FUNCTION "Gest Automatico" : VOID
TITLE =GESTIONE AUTOMATICO
AUTHOR : MassimoZ
VERSION : 0.1

BEGIN
NETWORK
TITLE ======== Automatico Barra 1 =======

NETWORK
TITLE =Aux Emergenze Macchine Barra 1 Intervenuta
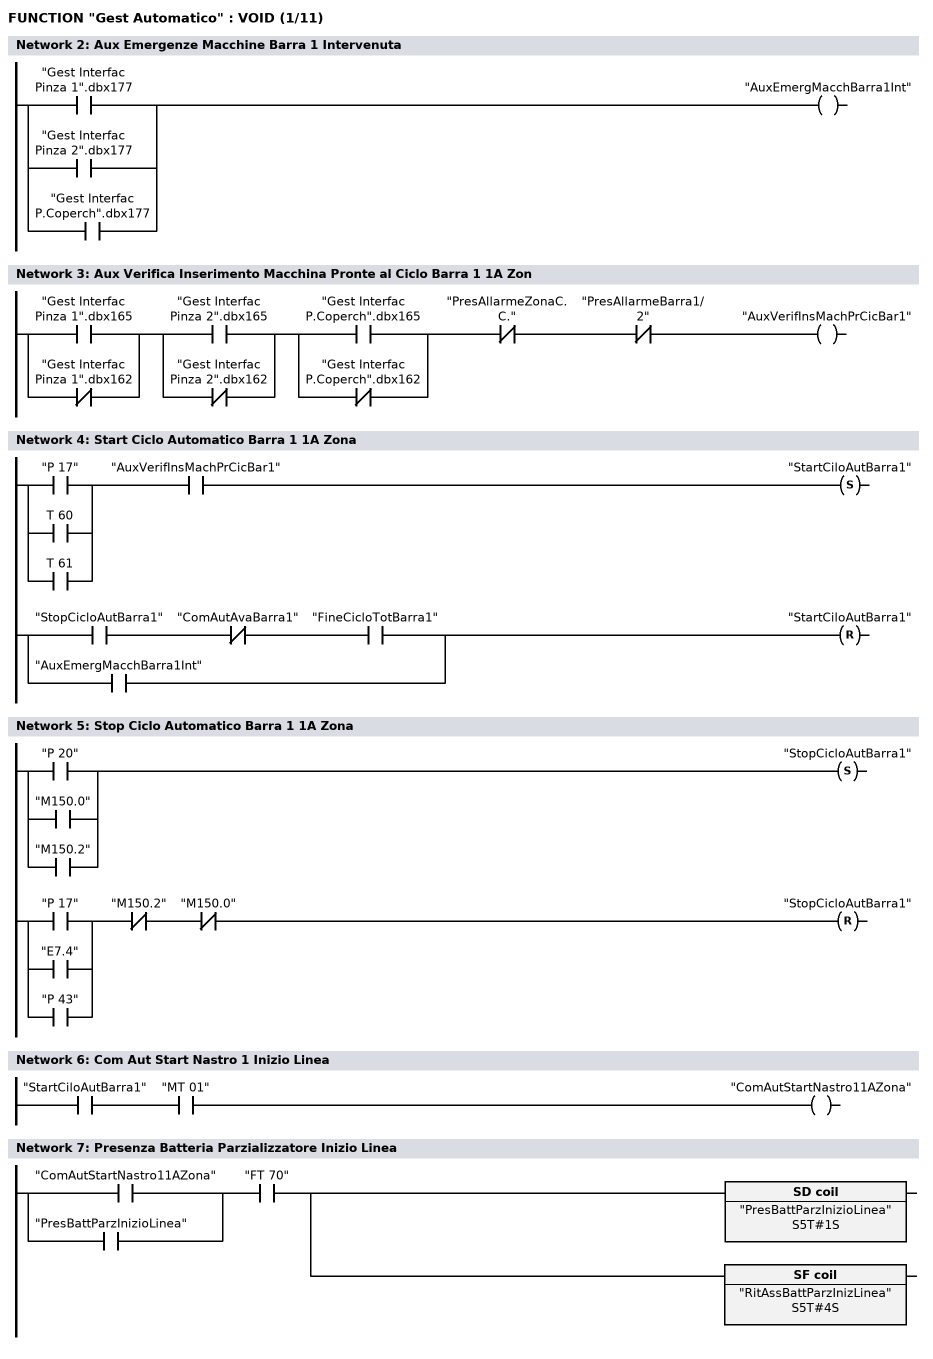
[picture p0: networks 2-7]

      O     "Gest Interfac Pinza 1".dbx177;
      O     "Gest Interfac Pinza 2".dbx177;
      O     "Gest Interfac P.Coperch".dbx177;
      =     "AuxEmergMacchBarra1Int";
NETWORK
TITLE =Aux Verifica Inserimento Macchina Pronte al Ciclo Barra 1 1A Zon

      U(    ;
      O     "Gest Interfac Pinza 1".dbx165;
      ON    "Gest Interfac Pinza 1".dbx162;
      )     ;
      U(    ;
      O     "Gest Interfac Pinza 2".dbx165;
      ON    "Gest Interfac Pinza 2".dbx162;
      )     ;
      U(    ;
      O     "Gest Interfac P.Coperch".dbx165;
      ON    "Gest Interfac P.Coperch".dbx162;
      )     ;
      UN    "PresAllarmeZonaC.C.";
      UN    "PresAllarmeBarra1/2";
      =     "AuxVerifInsMachPrCicBar1";
NETWORK
TITLE =Start Ciclo Automatico Barra 1 1A Zona

      U(    ;
      O     "P 17";
      O     T     60;
      O     T     61;
      )     ;
      U     "AuxVerifInsMachPrCicBar1";
      S     "StartCiloAutBarra1";
      U(    ;
      U     "StopCicloAutBarra1";
      UN    "ComAutAvaBarra1";
      U     "FineCicloTotBarra1";
      O     "AuxEmergMacchBarra1Int";
      )     ;
      R     "StartCiloAutBarra1";
      NOP   0;
NETWORK
TITLE =Stop Ciclo Automatico Barra 1 1A Zona

      U(    ;
      O     "P 20";
      O     "M150.0";
      O     "M150.2";
      )     ;
      S     "StopCicloAutBarra1";
      U(    ;
      O     "P 17";
      O     "E7.4";
      O     "P 43";
      )     ;
      UN    "M150.2";
      UN    "M150.0";
      R     "StopCicloAutBarra1";
      NOP   0;
NETWORK
TITLE =Com Aut Start Nastro 1 Inizio Linea

      U     "StartCiloAutBarra1";
      U     "MT 01";
      =     "ComAutStartNastro11AZona";
NETWORK
TITLE =Presenza Batteria Parzializzatore Inizio Linea

      U(    ;
      O     "ComAutStartNastro11AZona";
      O     "PresBattParzInizioLinea";
      )     ;
      U     "FT 70";
      L     S5T#1S;
      SE    "PresBattParzInizioLinea";
      L     S5T#4S;
      SA    "RitAssBattParzInizLinea";
NETWORK
TITLE =Verifica Mancanza Batteria su Parzializzatore Inizio Linea
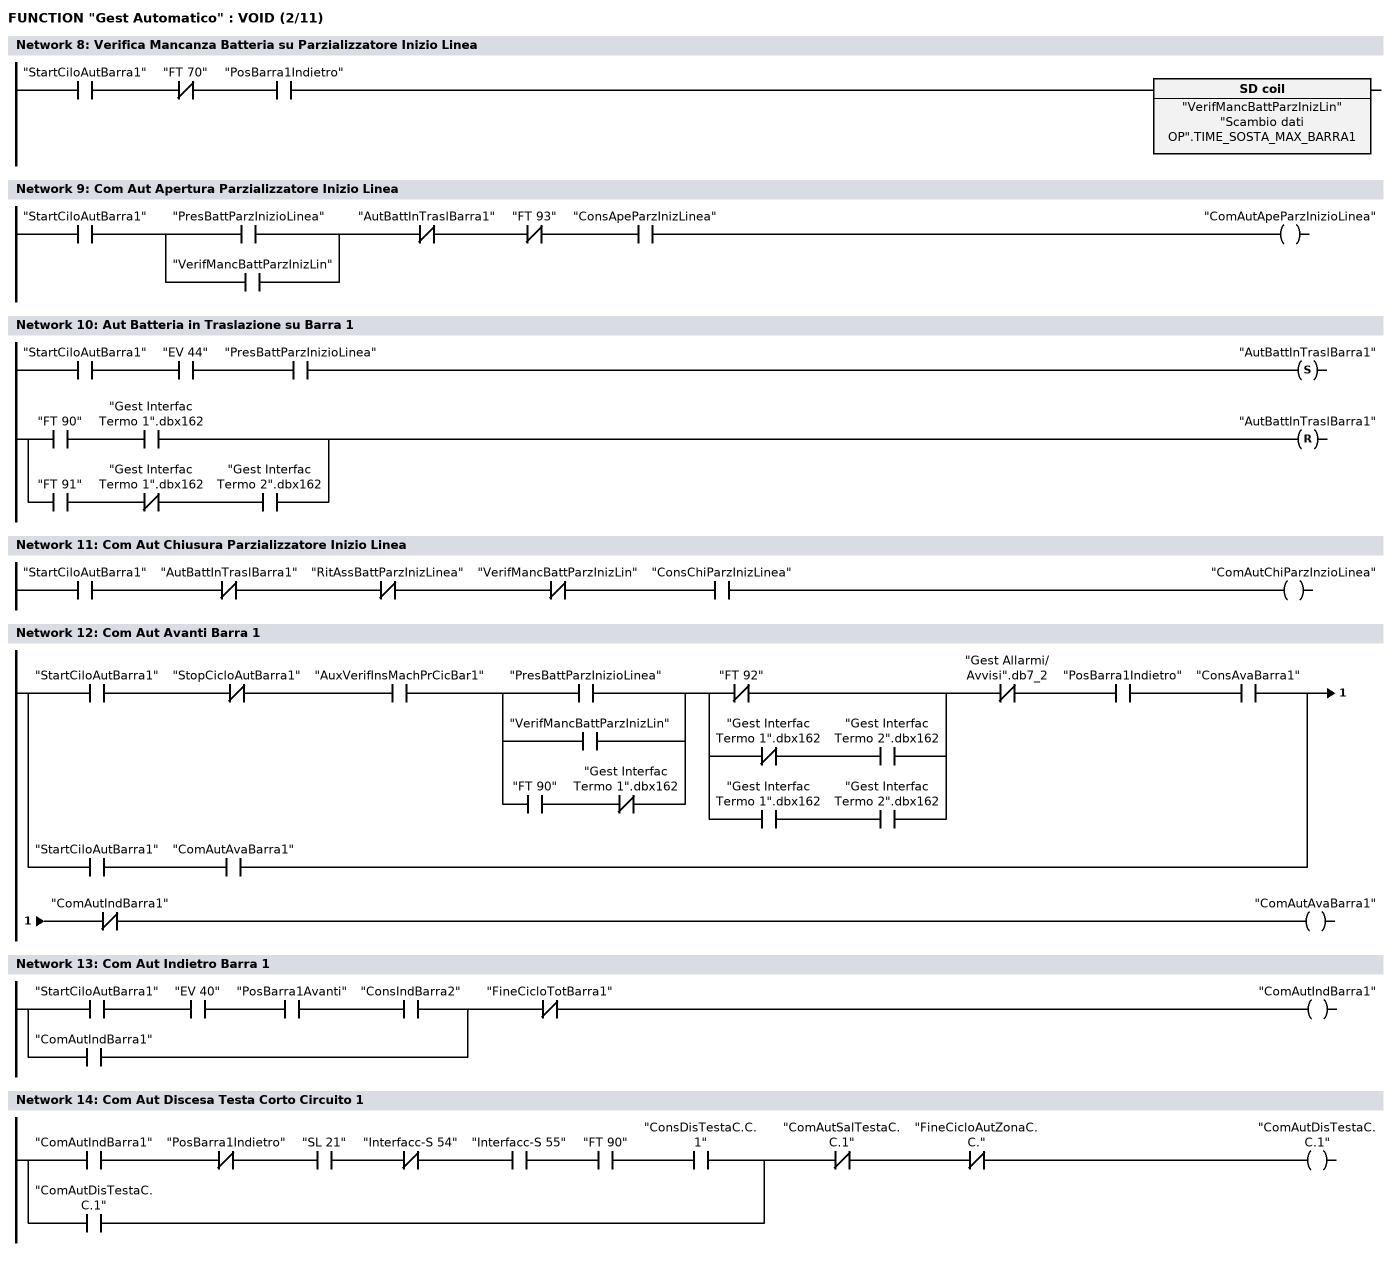
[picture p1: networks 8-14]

      U     "StartCiloAutBarra1";
      UN    "FT 70";
      U     "PosBarra1Indietro";
      L     "Scambio dati OP".TIME_SOSTA_MAX_BARRA1;
      SE    "VerifMancBattParzInizLin";
NETWORK
TITLE =Com Aut Apertura Parzializzatore Inizio Linea

      U     "StartCiloAutBarra1";
      U(    ;
      O     "PresBattParzInizioLinea";
      O     "VerifMancBattParzInizLin";
      )     ;
      UN    "AutBattInTraslBarra1";
      UN    "FT 93";
      U     "ConsApeParzInizLinea";
      =     "ComAutApeParzInizioLinea";
NETWORK
TITLE =Aut Batteria in Traslazione su Barra 1

      U     "StartCiloAutBarra1";
      U     "EV 44";
      U     "PresBattParzInizioLinea";
      S     "AutBattInTraslBarra1";
      U(    ;
      U     "FT 90";
      U     "Gest Interfac Termo 1".dbx162;
      O     ;
      U     "FT 91";
      UN    "Gest Interfac Termo 1".dbx162;
      U     "Gest Interfac Termo 2".dbx162;
      )     ;
      R     "AutBattInTraslBarra1";
      NOP   0;
NETWORK
TITLE =Com Aut Chiusura Parzializzatore Inizio Linea

      U     "StartCiloAutBarra1";
      UN    "AutBattInTraslBarra1";
      UN    "RitAssBattParzInizLinea";
      UN    "VerifMancBattParzInizLin";
      U     "ConsChiParzInizLinea";
      =     "ComAutChiParzInzioLinea";
NETWORK
TITLE =Com Aut Avanti Barra 1

      U(    ;
      U     "StartCiloAutBarra1";
      UN    "StopCicloAutBarra1";
      U     "AuxVerifInsMachPrCicBar1";
      U(    ;
      O     "PresBattParzInizioLinea";
      O     "VerifMancBattParzInizLin";
      O     ;
      U     "FT 90";
      UN    "Gest Interfac Termo 1".dbx162;
      )     ;
      U(    ;
      ON    "FT 92";
      O     ;
      UN    "Gest Interfac Termo 1".dbx162;
      U     "Gest Interfac Termo 2".dbx162;
      O     ;
      U     "Gest Interfac Termo 1".dbx162;
      U     "Gest Interfac Termo 2".dbx162;
      )     ;
      UN    "Gest Allarmi/Avvisi".db7_2;
      U     "PosBarra1Indietro";
      U     "ConsAvaBarra1";
      O     ;
      U     "StartCiloAutBarra1";
      U     "ComAutAvaBarra1";
      )     ;
      UN    "ComAutIndBarra1";
      =     "ComAutAvaBarra1";
NETWORK
TITLE =Com Aut Indietro Barra 1

      U(    ;
      U     "StartCiloAutBarra1";
      U     "EV 40";
      U     "PosBarra1Avanti";
      U     "ConsIndBarra2";
      O     "ComAutIndBarra1";
      )     ;
      UN    "FineCicloTotBarra1";
      =     "ComAutIndBarra1";
NETWORK
TITLE =Com Aut Discesa Testa Corto Circuito 1

      U(    ;
      U     "ComAutIndBarra1";
      UN    "PosBarra1Indietro";
      U     "SL 21";
      UN    "Interfacc-S 54";
      U     "Interfacc-S 55";
      U     "FT 90";
      U     "ConsDisTestaC.C.1";
      O     "ComAutDisTestaC.C.1";
      )     ;
      UN    "ComAutSalTestaC.C.1";
      UN    "FineCicloAutZonaC.C.";
      =     "ComAutDisTestaC.C.1";
NETWORK
TITLE =Com Aut Start Corto Circuito 1
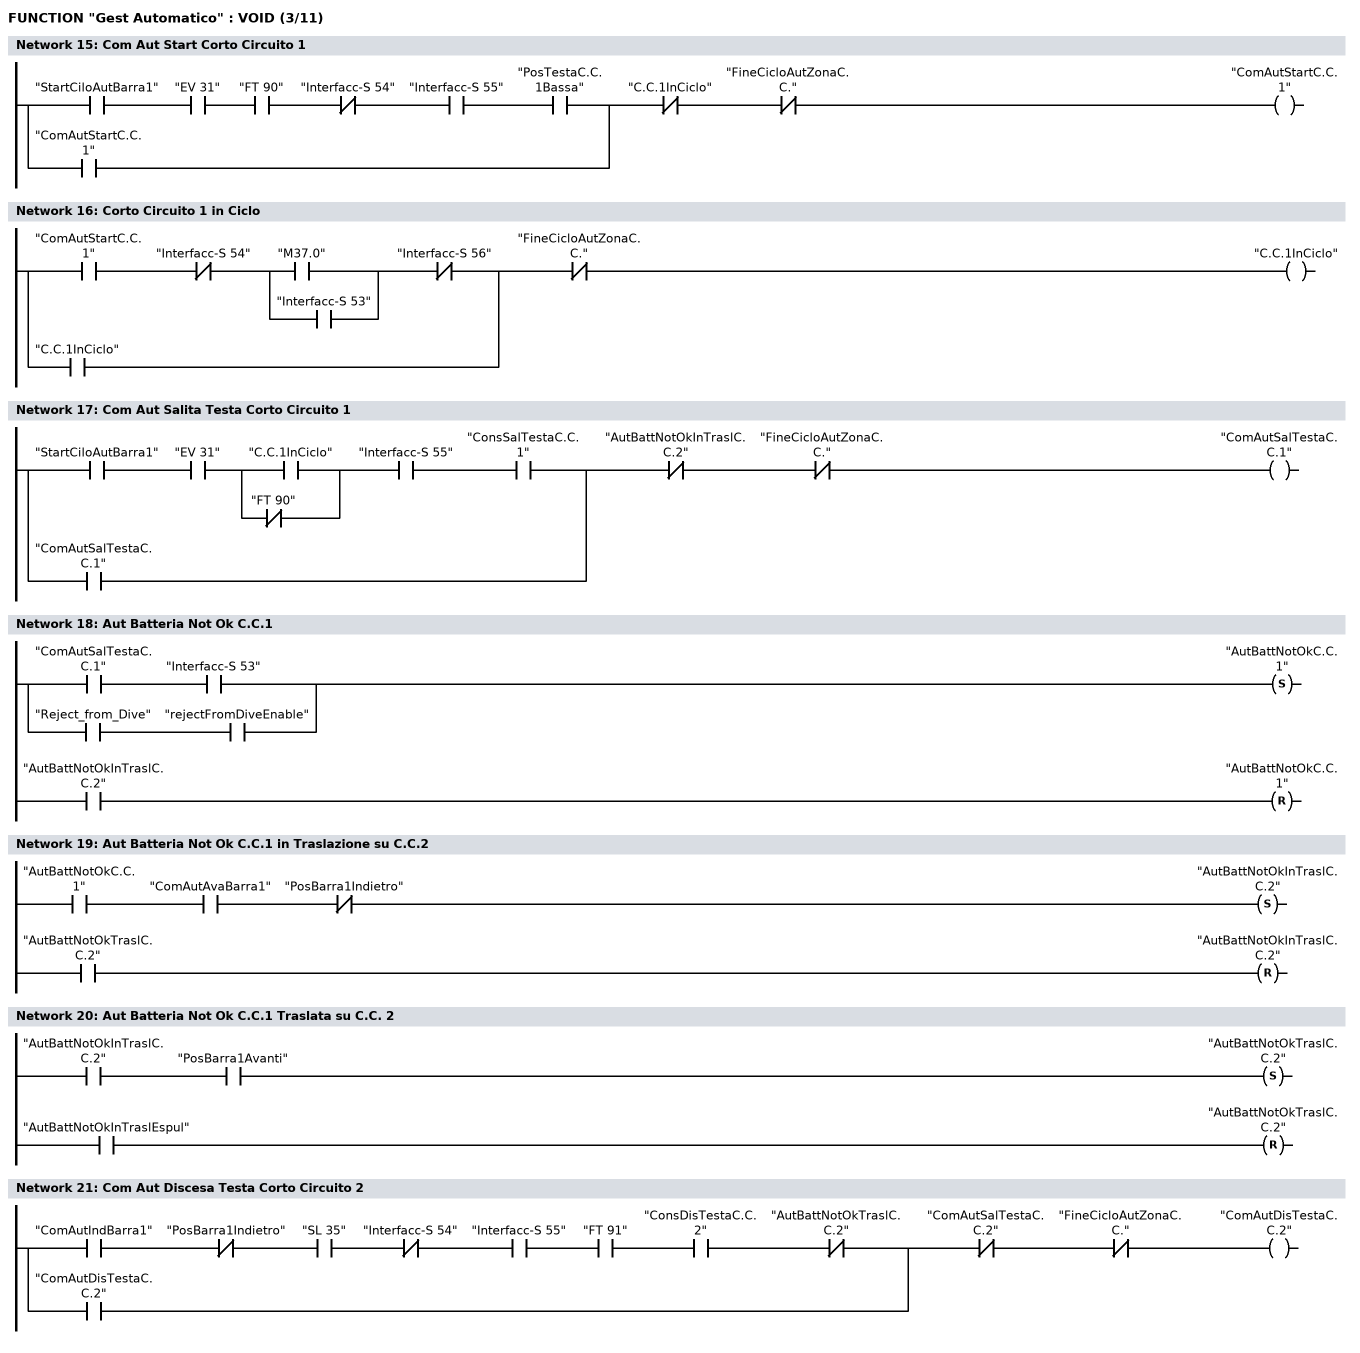
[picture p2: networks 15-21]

      U(    ;
      U     "StartCiloAutBarra1";
      U     "EV 31";
      U     "FT 90";
      UN    "Interfacc-S 54";
      U     "Interfacc-S 55";
      U     "PosTestaC.C.1Bassa";
      O     "ComAutStartC.C.1";
      )     ;
      UN    "C.C.1InCiclo";
      UN    "FineCicloAutZonaC.C.";
      =     "ComAutStartC.C.1";
NETWORK
TITLE =Corto Circuito 1 in Ciclo

      U(    ;
      U     "ComAutStartC.C.1";
      UN    "Interfacc-S 54";
      U(    ;
      O     "M37.0";
      O     "Interfacc-S 53";
      )     ;
      UN    "Interfacc-S 56";
      O     "C.C.1InCiclo";
      )     ;
      UN    "FineCicloAutZonaC.C.";
      =     "C.C.1InCiclo";
NETWORK
TITLE =Com Aut Salita Testa Corto Circuito 1

      U(    ;
      U     "StartCiloAutBarra1";
      U     "EV 31";
      U(    ;
      O     "C.C.1InCiclo";
      ON    "FT 90";
      )     ;
      U     "Interfacc-S 55";
      U     "ConsSalTestaC.C.1";
      O     "ComAutSalTestaC.C.1";
      )     ;
      UN    "AutBattNotOkInTraslC.C.2";
      UN    "FineCicloAutZonaC.C.";
      =     "ComAutSalTestaC.C.1";
NETWORK
TITLE =Aut Batteria Not Ok C.C.1

      U(    ;
      U     "ComAutSalTestaC.C.1";
      U     "Interfacc-S 53";
      O     ;
      U     "Reject_from_Dive";
      U     "rejectFromDiveEnable";
      )     ;
      S     "AutBattNotOkC.C.1";
      U     "AutBattNotOkInTraslC.C.2";
      R     "AutBattNotOkC.C.1";
      NOP   0;
NETWORK
TITLE =Aut Batteria Not Ok C.C.1 in Traslazione su C.C.2

      U     "AutBattNotOkC.C.1";
      U     "ComAutAvaBarra1";
      UN    "PosBarra1Indietro";
      S     "AutBattNotOkInTraslC.C.2";
      U     "AutBattNotOkTraslC.C.2";
      R     "AutBattNotOkInTraslC.C.2";
      NOP   0;
NETWORK
TITLE =Aut Batteria Not Ok C.C.1 Traslata su C.C. 2

      U     "AutBattNotOkInTraslC.C.2";
      U     "PosBarra1Avanti";
      S     "AutBattNotOkTraslC.C.2";
      U     "AutBattNotOkInTraslEspul";
      R     "AutBattNotOkTraslC.C.2";
      NOP   0;
NETWORK
TITLE =Com Aut Discesa Testa Corto Circuito 2

      U(    ;
      U     "ComAutIndBarra1";
      UN    "PosBarra1Indietro";
      U     "SL 35";
      UN    "Interfacc-S 54";
      U     "Interfacc-S 55";
      U     "FT 91";
      U     "ConsDisTestaC.C.2";
      UN    "AutBattNotOkTraslC.C.2";
      O     "ComAutDisTestaC.C.2";
      )     ;
      UN    "ComAutSalTestaC.C.2";
      UN    "FineCicloAutZonaC.C.";
      =     "ComAutDisTestaC.C.2";
NETWORK
TITLE =Com Aut Start Corto Circuito 2
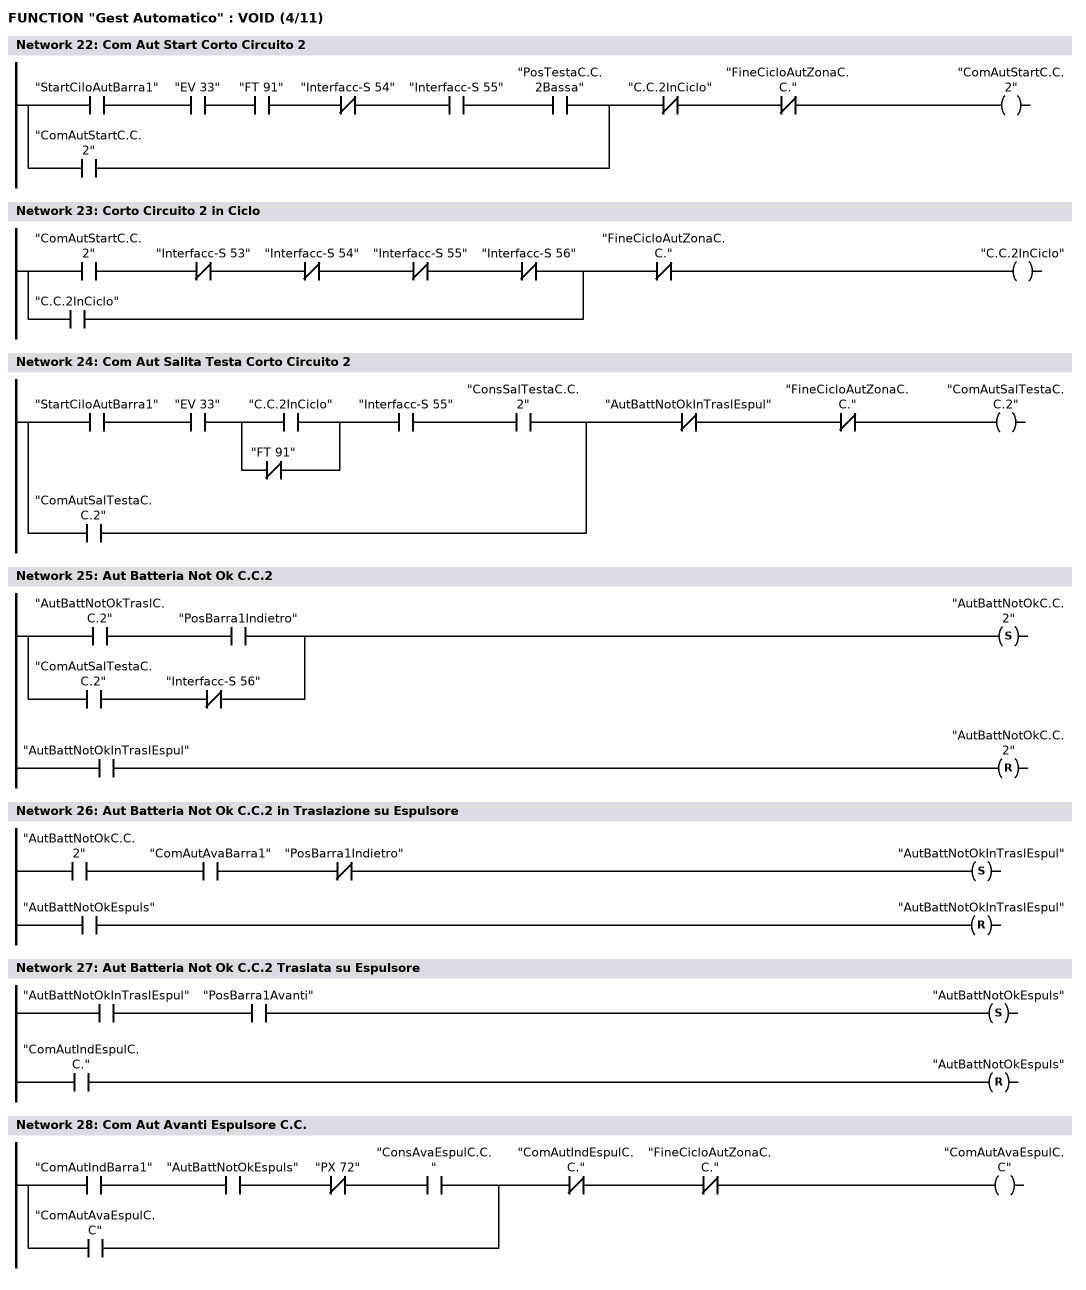
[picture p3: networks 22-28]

      U(    ;
      U     "StartCiloAutBarra1";
      U     "EV 33";
      U     "FT 91";
      UN    "Interfacc-S 54";
      U     "Interfacc-S 55";
      U     "PosTestaC.C.2Bassa";
      O     "ComAutStartC.C.2";
      )     ;
      UN    "C.C.2InCiclo";
      UN    "FineCicloAutZonaC.C.";
      =     "ComAutStartC.C.2";
NETWORK
TITLE =Corto Circuito 2 in Ciclo

      U(    ;
      U     "ComAutStartC.C.2";
      UN    "Interfacc-S 53";
      UN    "Interfacc-S 54";
      UN    "Interfacc-S 55";
      UN    "Interfacc-S 56";
      O     "C.C.2InCiclo";
      )     ;
      UN    "FineCicloAutZonaC.C.";
      =     "C.C.2InCiclo";
NETWORK
TITLE =Com Aut Salita Testa Corto Circuito 2

      U(    ;
      U     "StartCiloAutBarra1";
      U     "EV 33";
      U(    ;
      O     "C.C.2InCiclo";
      ON    "FT 91";
      )     ;
      U     "Interfacc-S 55";
      U     "ConsSalTestaC.C.2";
      O     "ComAutSalTestaC.C.2";
      )     ;
      UN    "AutBattNotOkInTraslEspul";
      UN    "FineCicloAutZonaC.C.";
      =     "ComAutSalTestaC.C.2";
NETWORK
TITLE =Aut Batteria Not Ok C.C.2

      U(    ;
      U     "AutBattNotOkTraslC.C.2";
      U     "PosBarra1Indietro";
      O     ;
      U     "ComAutSalTestaC.C.2";
      UN    "Interfacc-S 56";
      )     ;
      S     "AutBattNotOkC.C.2";
      U     "AutBattNotOkInTraslEspul";
      R     "AutBattNotOkC.C.2";
      NOP   0;
NETWORK
TITLE =Aut Batteria Not Ok C.C.2 in Traslazione su Espulsore

      U     "AutBattNotOkC.C.2";
      U     "ComAutAvaBarra1";
      UN    "PosBarra1Indietro";
      S     "AutBattNotOkInTraslEspul";
      U     "AutBattNotOkEspuls";
      R     "AutBattNotOkInTraslEspul";
      NOP   0;
NETWORK
TITLE =Aut Batteria Not Ok C.C.2 Traslata su Espulsore

      U     "AutBattNotOkInTraslEspul";
      U     "PosBarra1Avanti";
      S     "AutBattNotOkEspuls";
      U     "ComAutIndEspulC.C.";
      R     "AutBattNotOkEspuls";
      NOP   0;
NETWORK
TITLE =Com Aut Avanti Espulsore C.C.

      U(    ;
      U     "ComAutIndBarra1";
      U     "AutBattNotOkEspuls";
      UN    "PX 72";
      U     "ConsAvaEspulC.C.";
      O     "ComAutAvaEspulC.C";
      )     ;
      UN    "ComAutIndEspulC.C.";
      UN    "FineCicloAutZonaC.C.";
      =     "ComAutAvaEspulC.C";
NETWORK
TITLE =Com Aut Indietro Espulsore C.C.
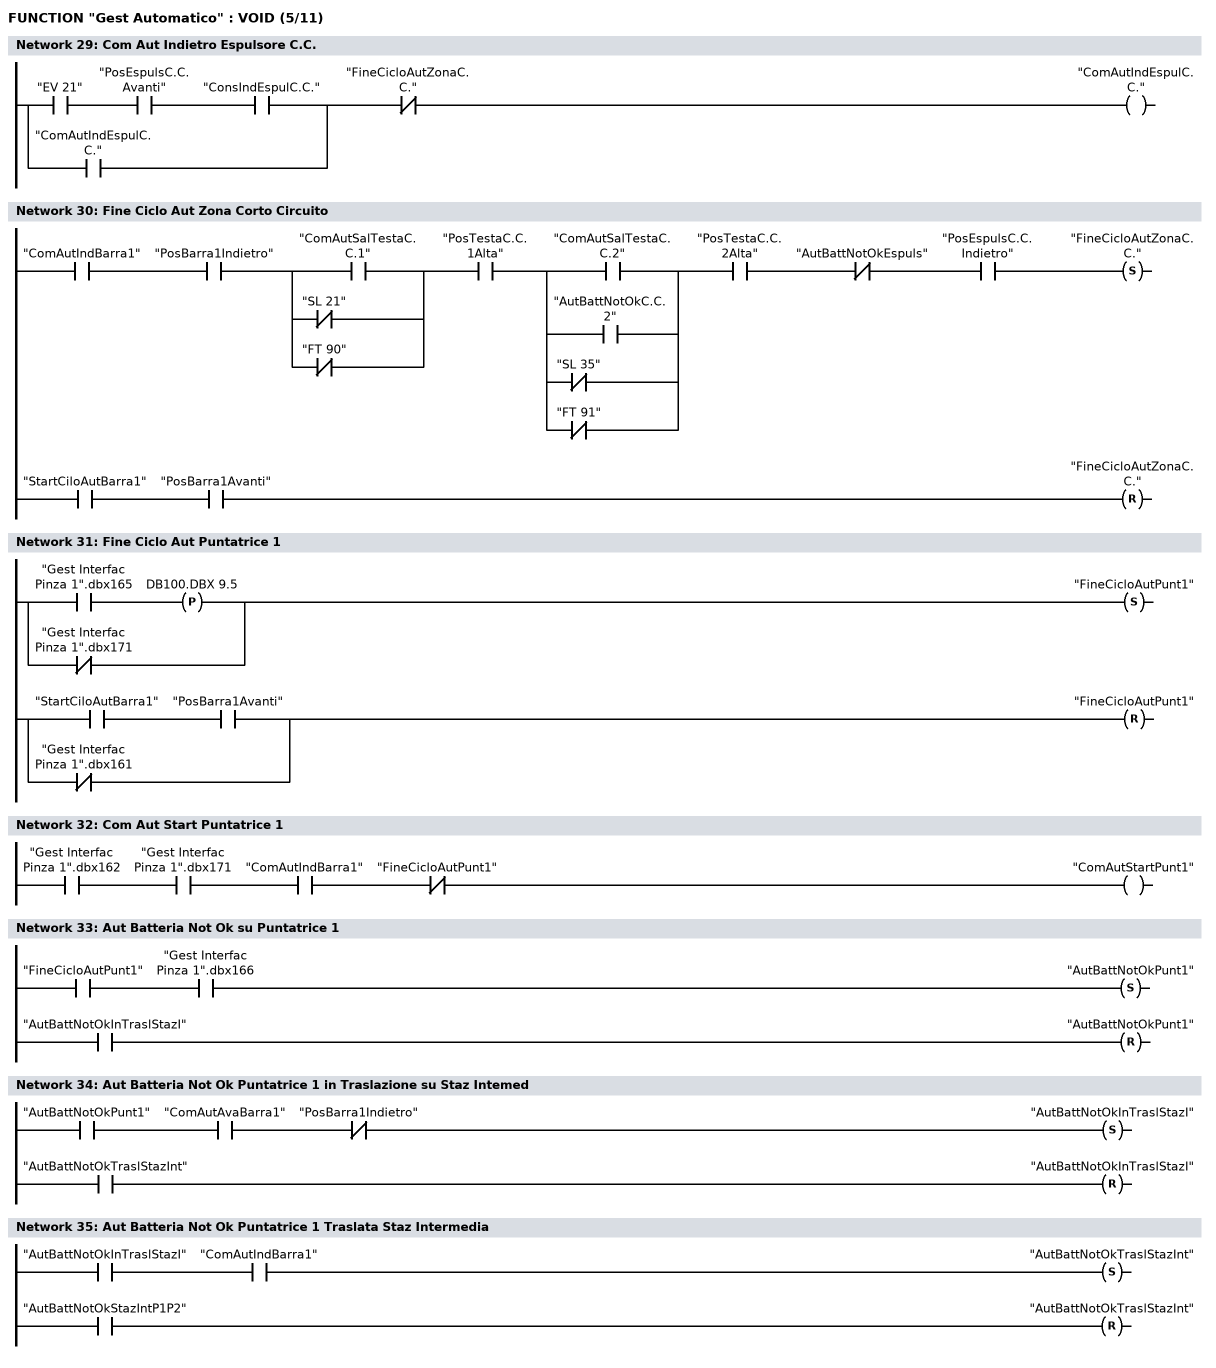
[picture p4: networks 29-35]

      U(    ;
      U     "EV 21";
      U     "PosEspulsC.C.Avanti";
      U     "ConsIndEspulC.C.";
      O     "ComAutIndEspulC.C.";
      )     ;
      UN    "FineCicloAutZonaC.C.";
      =     "ComAutIndEspulC.C.";
NETWORK
TITLE =Fine Ciclo Aut Zona Corto Circuito

      U     "ComAutIndBarra1";
      U     "PosBarra1Indietro";
      U(    ;
      O     "ComAutSalTestaC.C.1";
      ON    "SL 21";
      ON    "FT 90";
      )     ;
      U     "PosTestaC.C.1Alta";
      U(    ;
      O     "ComAutSalTestaC.C.2";
      O     "AutBattNotOkC.C.2";
      ON    "SL 35";
      ON    "FT 91";
      )     ;
      U     "PosTestaC.C.2Alta";
      UN    "AutBattNotOkEspuls";
      U     "PosEspulsC.C.Indietro";
      S     "FineCicloAutZonaC.C.";
      U     "StartCiloAutBarra1";
      U     "PosBarra1Avanti";
      R     "FineCicloAutZonaC.C.";
      NOP   0;
NETWORK
TITLE =Fine Ciclo Aut Puntatrice 1

      U(    ;
      U     "Gest Interfac Pinza 1".dbx165;
      FP    DB100.DBX    9.5;
      ON    "Gest Interfac Pinza 1".dbx171;
      )     ;
      S     "FineCicloAutPunt1";
      U(    ;
      U     "StartCiloAutBarra1";
      U     "PosBarra1Avanti";
      ON    "Gest Interfac Pinza 1".dbx161;
      )     ;
      R     "FineCicloAutPunt1";
      NOP   0;
NETWORK
TITLE =Com Aut Start Puntatrice 1

      U     "Gest Interfac Pinza 1".dbx162;
      U     "Gest Interfac Pinza 1".dbx171;
      U     "ComAutIndBarra1";
      UN    "FineCicloAutPunt1";
      =     "ComAutStartPunt1";
NETWORK
TITLE =Aut Batteria Not Ok su Puntatrice 1

      U     "FineCicloAutPunt1";
      U     "Gest Interfac Pinza 1".dbx166;
      S     "AutBattNotOkPunt1";
      U     "AutBattNotOkInTraslStazI";
      R     "AutBattNotOkPunt1";
      NOP   0;
NETWORK
TITLE =Aut Batteria Not Ok Puntatrice 1 in Traslazione su Staz Intemed

      U     "AutBattNotOkPunt1";
      U     "ComAutAvaBarra1";
      UN    "PosBarra1Indietro";
      S     "AutBattNotOkInTraslStazI";
      U     "AutBattNotOkTraslStazInt";
      R     "AutBattNotOkInTraslStazI";
      NOP   0;
NETWORK
TITLE =Aut Batteria Not Ok Puntatrice 1 Traslata Staz Intermedia

      U     "AutBattNotOkInTraslStazI";
      U     "ComAutIndBarra1";
      S     "AutBattNotOkTraslStazInt";
      U     "AutBattNotOkStazIntP1P2";
      R     "AutBattNotOkTraslStazInt";
      NOP   0;
NETWORK
TITLE =Aut Batteria Not Ok su Stazione Intermedia
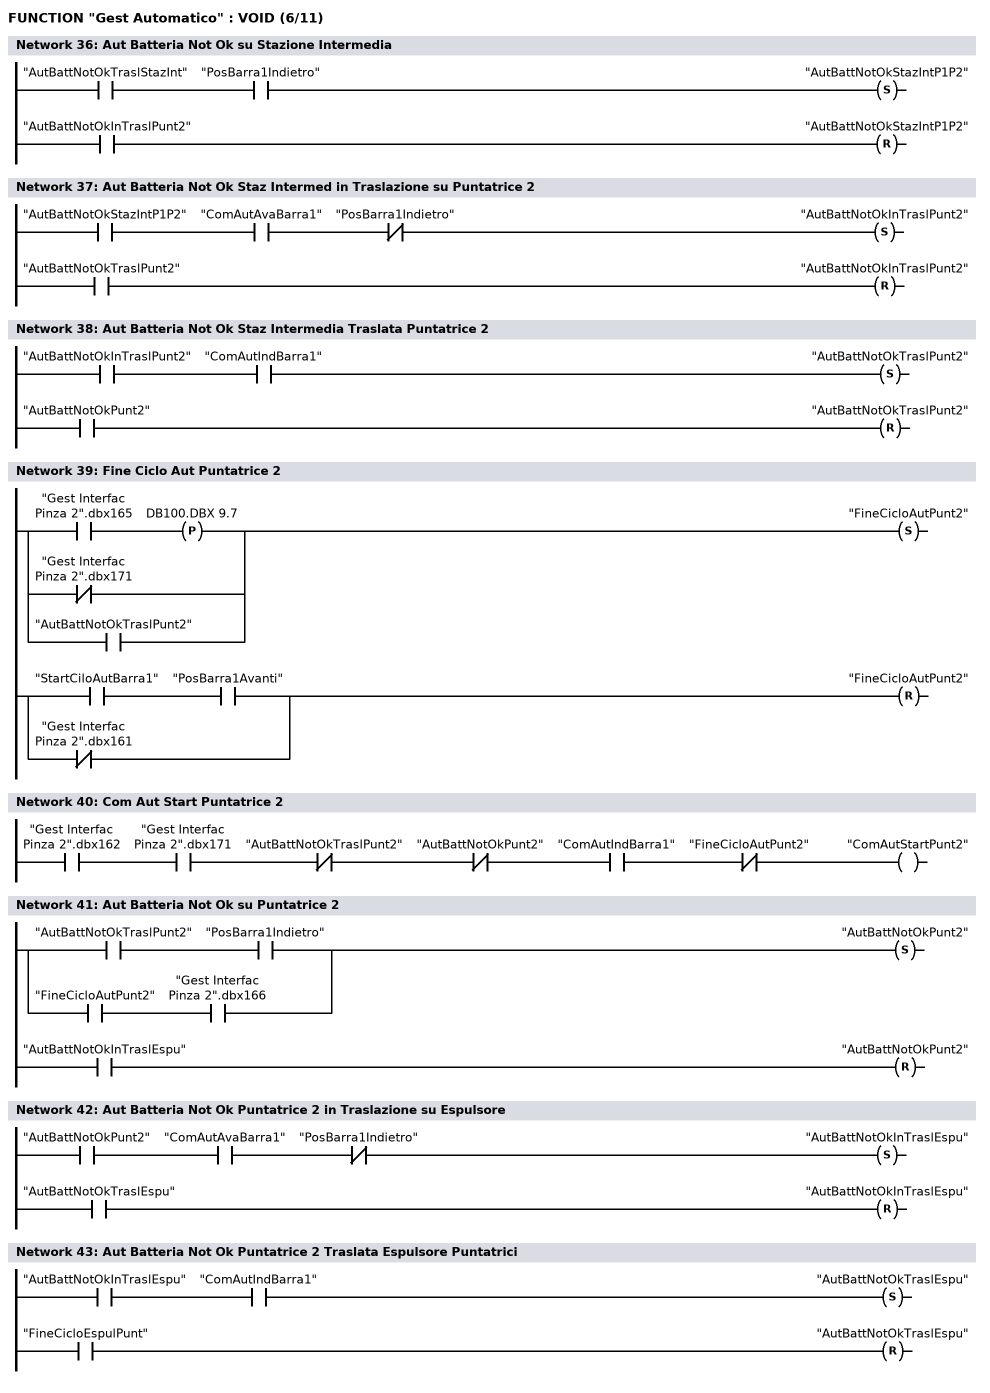
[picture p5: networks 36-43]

      U     "AutBattNotOkTraslStazInt";
      U     "PosBarra1Indietro";
      S     "AutBattNotOkStazIntP1P2";
      U     "AutBattNotOkInTraslPunt2";
      R     "AutBattNotOkStazIntP1P2";
      NOP   0;
NETWORK
TITLE =Aut Batteria Not Ok Staz Intermed in Traslazione su Puntatrice 2

      U     "AutBattNotOkStazIntP1P2";
      U     "ComAutAvaBarra1";
      UN    "PosBarra1Indietro";
      S     "AutBattNotOkInTraslPunt2";
      U     "AutBattNotOkTraslPunt2";
      R     "AutBattNotOkInTraslPunt2";
      NOP   0;
NETWORK
TITLE =Aut Batteria Not Ok Staz Intermedia Traslata Puntatrice 2

      U     "AutBattNotOkInTraslPunt2";
      U     "ComAutIndBarra1";
      S     "AutBattNotOkTraslPunt2";
      U     "AutBattNotOkPunt2";
      R     "AutBattNotOkTraslPunt2";
      NOP   0;
NETWORK
TITLE =Fine Ciclo Aut Puntatrice 2

      U(    ;
      U     "Gest Interfac Pinza 2".dbx165;
      FP    DB100.DBX    9.7;
      ON    "Gest Interfac Pinza 2".dbx171;
      O     "AutBattNotOkTraslPunt2";
      )     ;
      S     "FineCicloAutPunt2";
      U(    ;
      U     "StartCiloAutBarra1";
      U     "PosBarra1Avanti";
      ON    "Gest Interfac Pinza 2".dbx161;
      )     ;
      R     "FineCicloAutPunt2";
      NOP   0;
NETWORK
TITLE =Com Aut Start Puntatrice 2

      U     "Gest Interfac Pinza 2".dbx162;
      U     "Gest Interfac Pinza 2".dbx171;
      UN    "AutBattNotOkTraslPunt2";
      UN    "AutBattNotOkPunt2";
      U     "ComAutIndBarra1";
      UN    "FineCicloAutPunt2";
      =     "ComAutStartPunt2";
NETWORK
TITLE =Aut Batteria Not Ok su Puntatrice 2

      U(    ;
      U     "AutBattNotOkTraslPunt2";
      U     "PosBarra1Indietro";
      O     ;
      U     "FineCicloAutPunt2";
      U     "Gest Interfac Pinza 2".dbx166;
      )     ;
      S     "AutBattNotOkPunt2";
      U     "AutBattNotOkInTraslEspu";
      R     "AutBattNotOkPunt2";
      NOP   0;
NETWORK
TITLE =Aut Batteria Not Ok Puntatrice 2 in Traslazione su Espulsore

      U     "AutBattNotOkPunt2";
      U     "ComAutAvaBarra1";
      UN    "PosBarra1Indietro";
      S     "AutBattNotOkInTraslEspu";
      U     "AutBattNotOkTraslEspu";
      R     "AutBattNotOkInTraslEspu";
      NOP   0;
NETWORK
TITLE =Aut Batteria Not Ok Puntatrice 2 Traslata Espulsore Puntatrici

      U     "AutBattNotOkInTraslEspu";
      U     "ComAutIndBarra1";
      S     "AutBattNotOkTraslEspu";
      U     "FineCicloEspulPunt";
      R     "AutBattNotOkTraslEspu";
      NOP   0;
NETWORK
TITLE =Fine Ciclo Espulsore Puntatrici
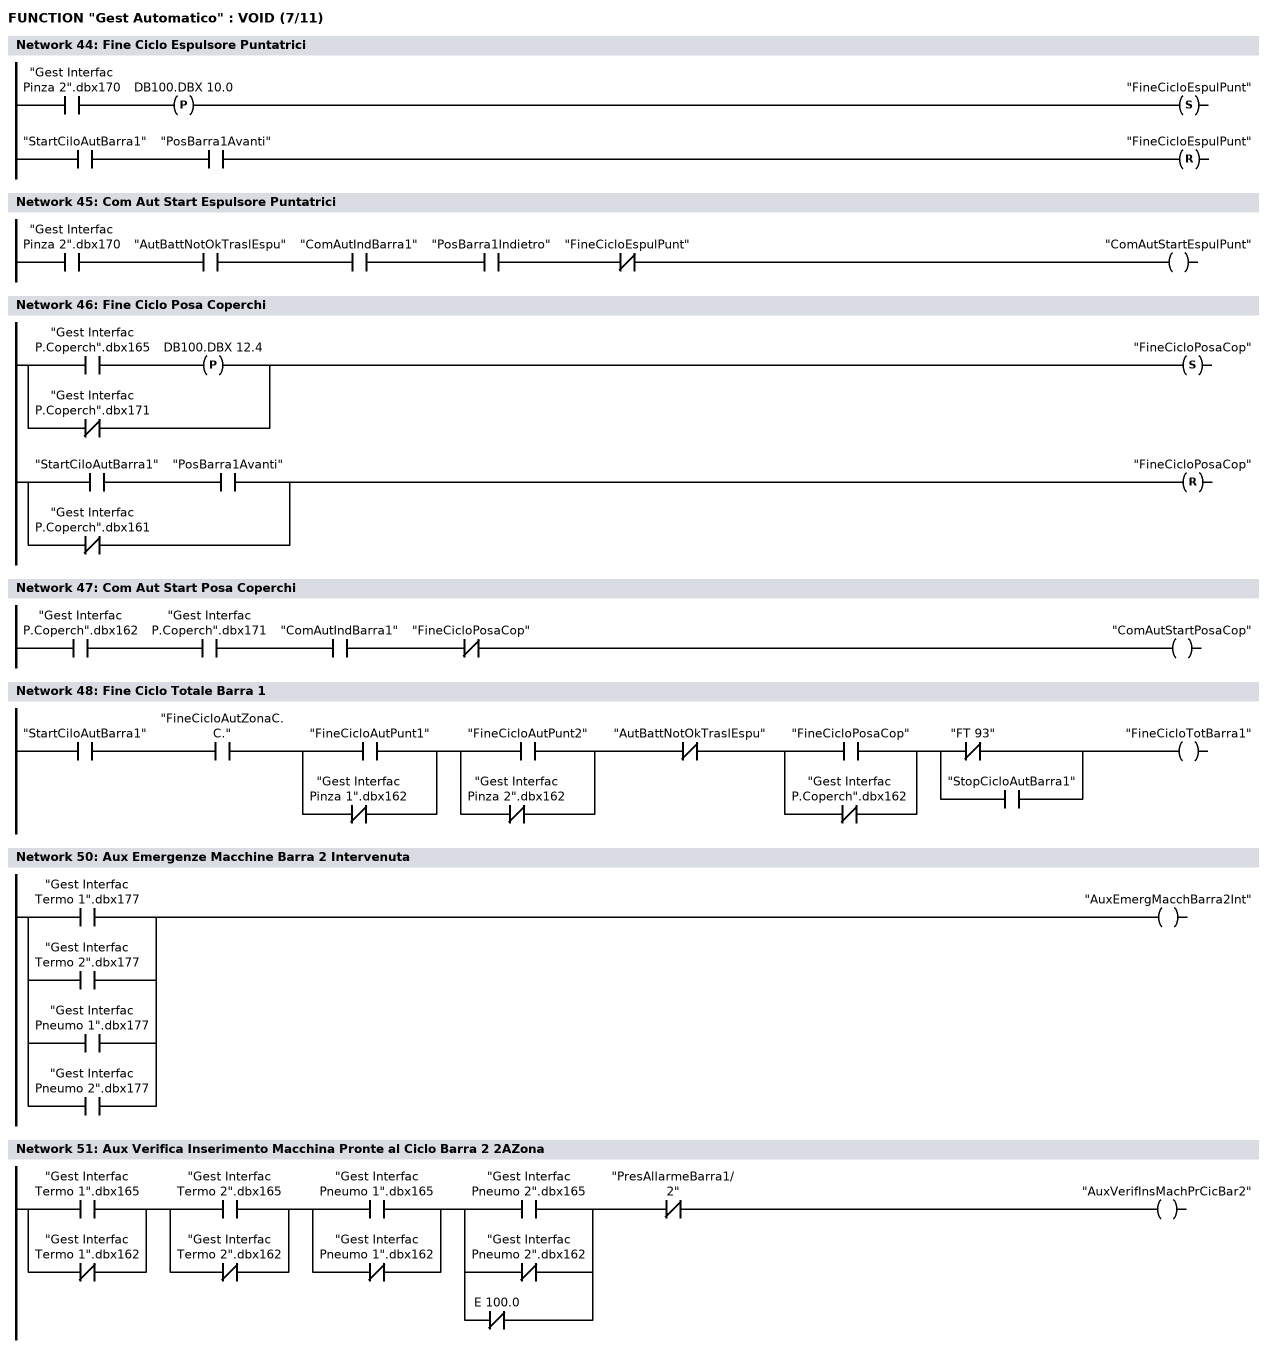
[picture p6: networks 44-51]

      U     "Gest Interfac Pinza 2".dbx170;
      FP    DB100.DBX   10.0;
      S     "FineCicloEspulPunt";
      U     "StartCiloAutBarra1";
      U     "PosBarra1Avanti";
      R     "FineCicloEspulPunt";
      NOP   0;
NETWORK
TITLE =Com Aut Start Espulsore Puntatrici

      U     "Gest Interfac Pinza 2".dbx170;
      U     "AutBattNotOkTraslEspu";
      U     "ComAutIndBarra1";
      U     "PosBarra1Indietro";
      UN    "FineCicloEspulPunt";
      =     "ComAutStartEspulPunt";
NETWORK
TITLE =Fine Ciclo Posa Coperchi

      U(    ;
      U     "Gest Interfac P.Coperch".dbx165;
      FP    DB100.DBX   12.4;
      ON    "Gest Interfac P.Coperch".dbx171;
      )     ;
      S     "FineCicloPosaCop";
      U(    ;
      U     "StartCiloAutBarra1";
      U     "PosBarra1Avanti";
      ON    "Gest Interfac P.Coperch".dbx161;
      )     ;
      R     "FineCicloPosaCop";
      NOP   0;
NETWORK
TITLE =Com Aut Start Posa Coperchi

      U     "Gest Interfac P.Coperch".dbx162;
      U     "Gest Interfac P.Coperch".dbx171;
      U     "ComAutIndBarra1";
      UN    "FineCicloPosaCop";
      =     "ComAutStartPosaCop";
NETWORK
TITLE =Fine Ciclo Totale Barra 1

      U     "StartCiloAutBarra1";
      U     "FineCicloAutZonaC.C.";
      U(    ;
      O     "FineCicloAutPunt1";
      ON    "Gest Interfac Pinza 1".dbx162;
      )     ;
      U(    ;
      O     "FineCicloAutPunt2";
      ON    "Gest Interfac Pinza 2".dbx162;
      )     ;
      UN    "AutBattNotOkTraslEspu";
      U(    ;
      O     "FineCicloPosaCop";
      ON    "Gest Interfac P.Coperch".dbx162;
      )     ;
      U(    ;
      ON    "FT 93";
      O     "StopCicloAutBarra1";
      )     ;
      =     "FineCicloTotBarra1";
NETWORK
TITLE ======== Automatico Barra 2 ========

NETWORK
TITLE =Aux Emergenze Macchine Barra 2 Intervenuta

      O     "Gest Interfac Termo 1".dbx177;
      O     "Gest Interfac Termo 2".dbx177;
      O     "Gest Interfac Pneumo 1".dbx177;
      O     "Gest Interfac Pneumo 2".dbx177;
      =     "AuxEmergMacchBarra2Int";
NETWORK
TITLE =Aux Verifica Inserimento Macchina Pronte al Ciclo Barra 2 2AZona

      U(    ;
      O     "Gest Interfac Termo 1".dbx165;
      ON    "Gest Interfac Termo 1".dbx162;
      )     ;
      U(    ;
      O     "Gest Interfac Termo 2".dbx165;
      ON    "Gest Interfac Termo 2".dbx162;
      )     ;
      U(    ;
      O     "Gest Interfac Pneumo 1".dbx165;
      ON    "Gest Interfac Pneumo 1".dbx162;
      )     ;
      U(    ;
      O     "Gest Interfac Pneumo 2".dbx165;
      ON    "Gest Interfac Pneumo 2".dbx162;
      ON    E    100.0;
      )     ;
      UN    "PresAllarmeBarra1/2";
      =     "AuxVerifInsMachPrCicBar2";
NETWORK
TITLE =Start Ciclo Automatico Barra 2 2A Zona
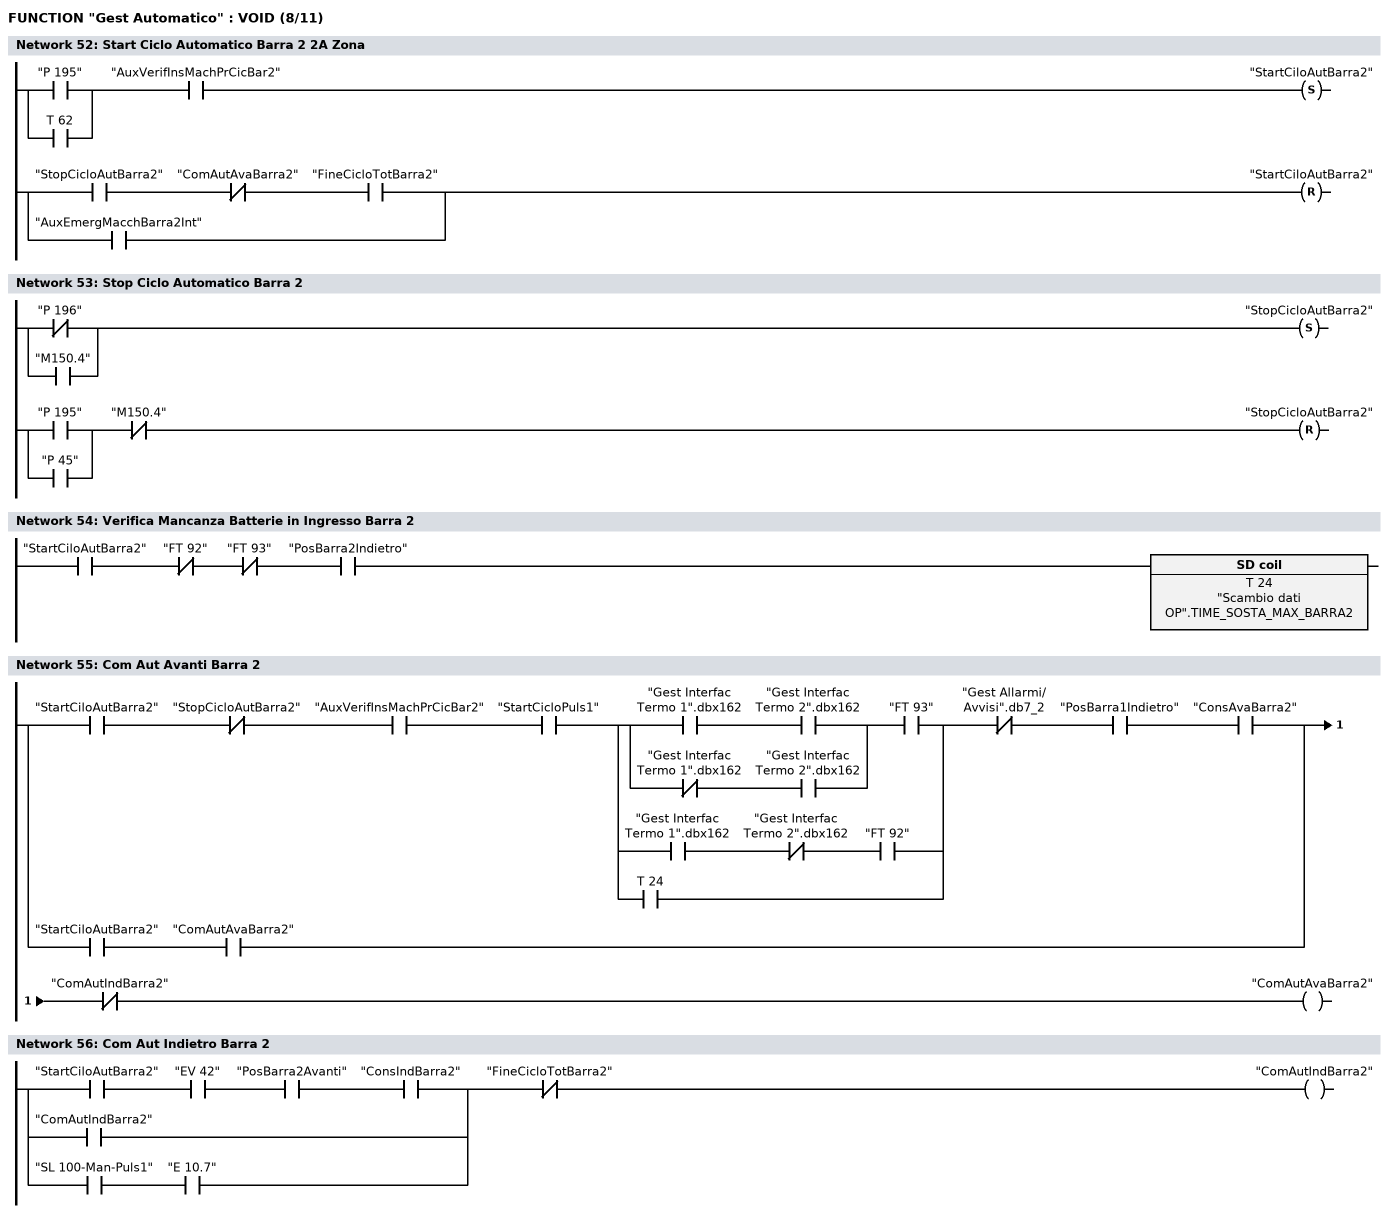
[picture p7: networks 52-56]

      U(    ;
      O     "P 195";
      O     T     62;
      )     ;
      U     "AuxVerifInsMachPrCicBar2";
      S     "StartCiloAutBarra2";
      U(    ;
      U     "StopCicloAutBarra2";
      UN    "ComAutAvaBarra2";
      U     "FineCicloTotBarra2";
      O     "AuxEmergMacchBarra2Int";
      )     ;
      R     "StartCiloAutBarra2";
      NOP   0;
NETWORK
TITLE =Stop Ciclo Automatico Barra 2

      U(    ;
      ON    "P 196";
      O     "M150.4";
      )     ;
      S     "StopCicloAutBarra2";
      U(    ;
      O     "P 195";
      O     "P 45";
      )     ;
      UN    "M150.4";
      R     "StopCicloAutBarra2";
      NOP   0;
NETWORK
TITLE =Verifica Mancanza Batterie in Ingresso Barra 2

      U     "StartCiloAutBarra2";
      UN    "FT 92";
      UN    "FT 93";
      U     "PosBarra2Indietro";
      L     "Scambio dati OP".TIME_SOSTA_MAX_BARRA2;
      SE    T     24;
NETWORK
TITLE =Com Aut Avanti Barra 2

      U(    ;
      U     "StartCiloAutBarra2";
      UN    "StopCicloAutBarra2";
      U     "AuxVerifInsMachPrCicBar2";
      U     "StartCicloPuls1";
      U(    ;
      U(    ;
      U     "Gest Interfac Termo 1".dbx162;
      U     "Gest Interfac Termo 2".dbx162;
      O     ;
      UN    "Gest Interfac Termo 1".dbx162;
      U     "Gest Interfac Termo 2".dbx162;
      )     ;
      U     "FT 93";
      O     ;
      U     "Gest Interfac Termo 1".dbx162;
      UN    "Gest Interfac Termo 2".dbx162;
      U     "FT 92";
      O     T     24;
      )     ;
      UN    "Gest Allarmi/Avvisi".db7_2;
      U     "PosBarra1Indietro";
      U     "ConsAvaBarra2";
      O     ;
      U     "StartCiloAutBarra2";
      U     "ComAutAvaBarra2";
      )     ;
      UN    "ComAutIndBarra2";
      =     "ComAutAvaBarra2";
NETWORK
TITLE =Com Aut Indietro Barra 2

      U(    ;
      U     "StartCiloAutBarra2";
      U     "EV 42";
      U     "PosBarra2Avanti";
      U     "ConsIndBarra2";
      O     "ComAutIndBarra2";
      O     ;
      U     "SL 100-Man-Puls1";
      U     "E      10.7";
      )     ;
      UN    "FineCicloTotBarra2";
      =     "ComAutIndBarra2";
NETWORK
TITLE =Fine Ciclo Termo 1
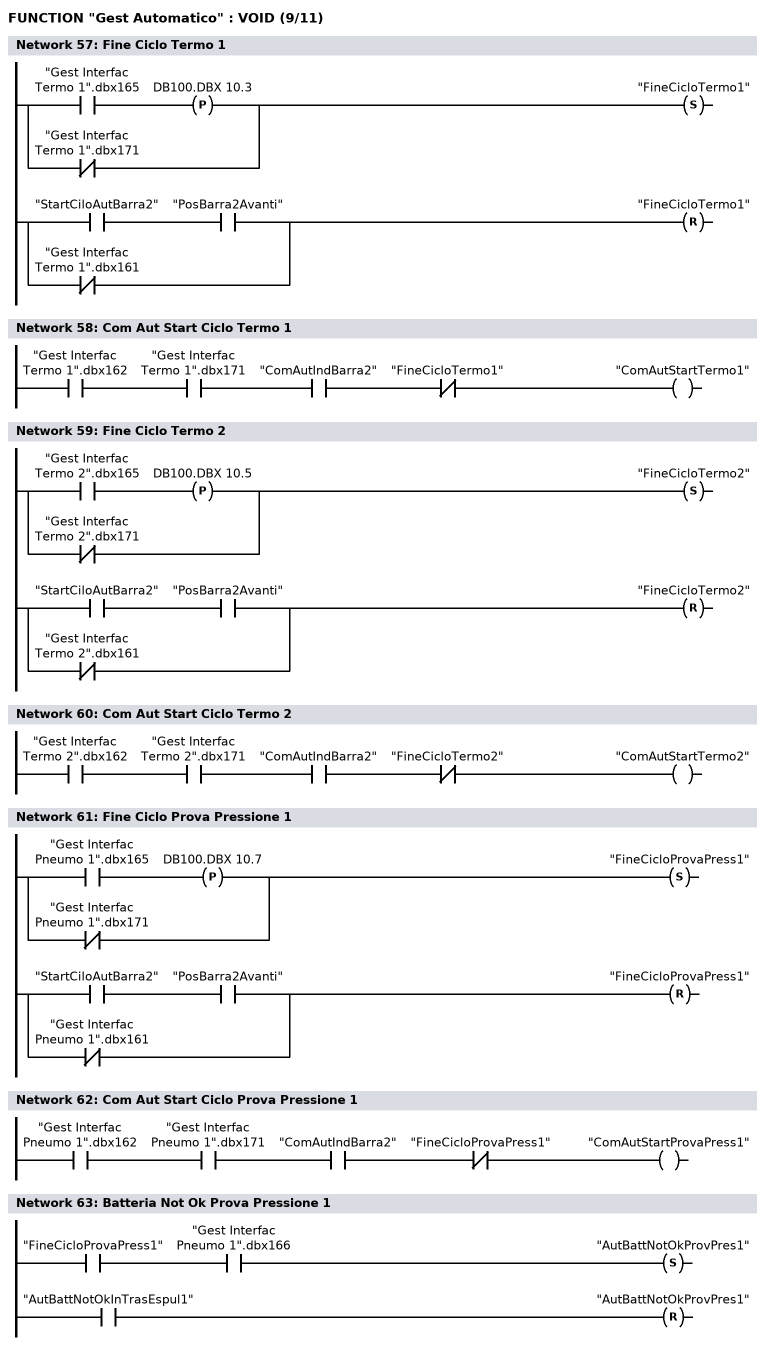
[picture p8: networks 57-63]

      U(    ;
      U     "Gest Interfac Termo 1".dbx165;
      FP    DB100.DBX   10.3;
      ON    "Gest Interfac Termo 1".dbx171;
      )     ;
      S     "FineCicloTermo1";
      U(    ;
      U     "StartCiloAutBarra2";
      U     "PosBarra2Avanti";
      ON    "Gest Interfac Termo 1".dbx161;
      )     ;
      R     "FineCicloTermo1";
      NOP   0;
NETWORK
TITLE =Com Aut Start Ciclo Termo 1

      U     "Gest Interfac Termo 1".dbx162;
      U     "Gest Interfac Termo 1".dbx171;
      U     "ComAutIndBarra2";
      UN    "FineCicloTermo1";
      =     "ComAutStartTermo1";
NETWORK
TITLE =Fine Ciclo Termo 2

      U(    ;
      U     "Gest Interfac Termo 2".dbx165;
      FP    DB100.DBX   10.5;
      ON    "Gest Interfac Termo 2".dbx171;
      )     ;
      S     "FineCicloTermo2";
      U(    ;
      U     "StartCiloAutBarra2";
      U     "PosBarra2Avanti";
      ON    "Gest Interfac Termo 2".dbx161;
      )     ;
      R     "FineCicloTermo2";
      NOP   0;
NETWORK
TITLE =Com Aut Start Ciclo Termo 2

      U     "Gest Interfac Termo 2".dbx162;
      U     "Gest Interfac Termo 2".dbx171;
      U     "ComAutIndBarra2";
      UN    "FineCicloTermo2";
      =     "ComAutStartTermo2";
NETWORK
TITLE =Fine Ciclo Prova Pressione 1

      U(    ;
      U     "Gest Interfac Pneumo 1".dbx165;
      FP    DB100.DBX   10.7;
      ON    "Gest Interfac Pneumo 1".dbx171;
      )     ;
      S     "FineCicloProvaPress1";
      U(    ;
      U     "StartCiloAutBarra2";
      U     "PosBarra2Avanti";
      ON    "Gest Interfac Pneumo 1".dbx161;
      )     ;
      R     "FineCicloProvaPress1";
      NOP   0;
NETWORK
TITLE =Com Aut Start Ciclo Prova Pressione 1

      U     "Gest Interfac Pneumo 1".dbx162;
      U     "Gest Interfac Pneumo 1".dbx171;
      U     "ComAutIndBarra2";
      UN    "FineCicloProvaPress1";
      =     "ComAutStartProvaPress1";
NETWORK
TITLE =Batteria Not Ok Prova Pressione 1

      U     "FineCicloProvaPress1";
      U     "Gest Interfac Pneumo 1".dbx166;
      S     "AutBattNotOkProvPres1";
      U     "AutBattNotOkInTrasEspul1";
      R     "AutBattNotOkProvPres1";
      NOP   0;
NETWORK
TITLE =Batteria Not Ok Prova Press.1 in Traslazione su Espulsore 1
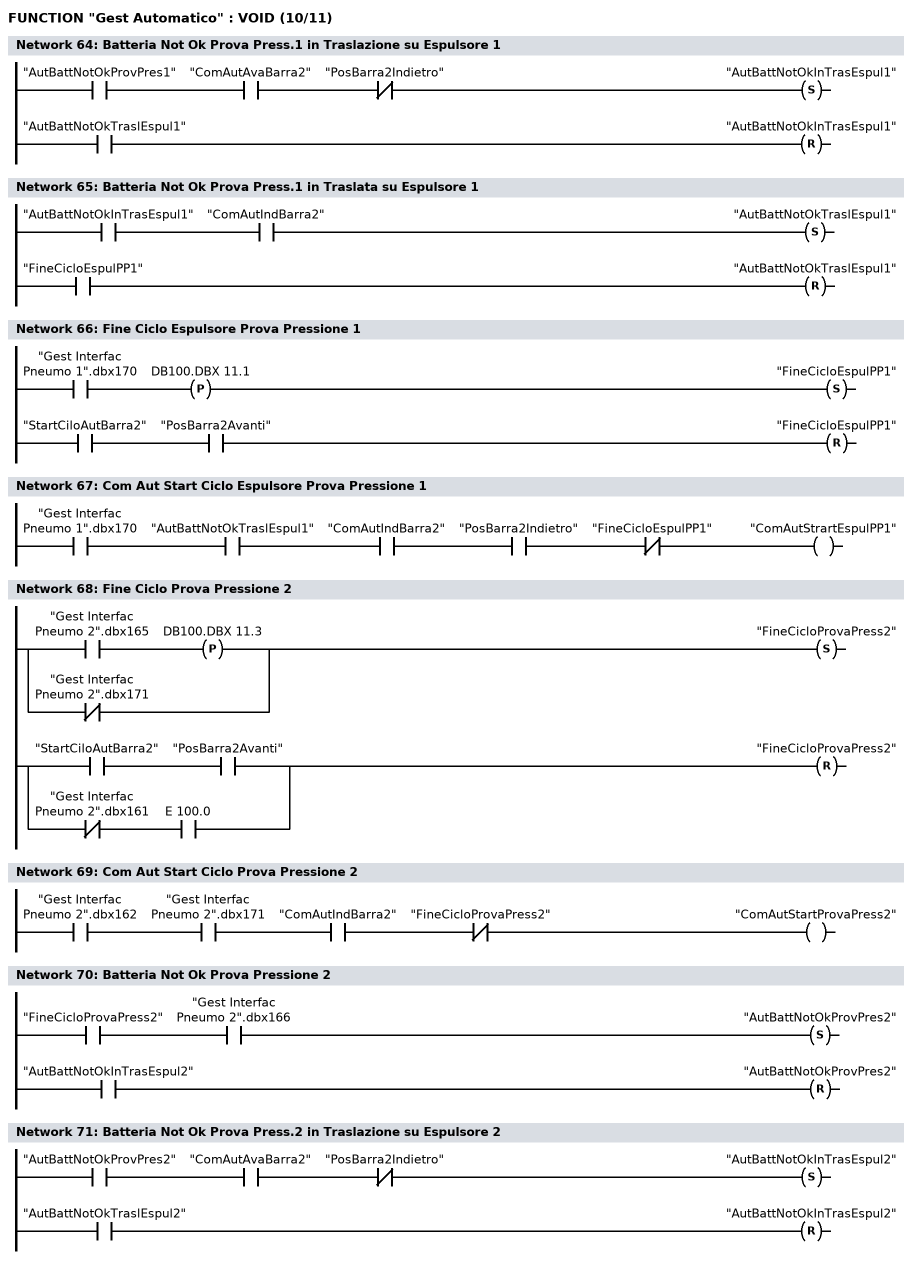
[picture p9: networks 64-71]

      U     "AutBattNotOkProvPres1";
      U     "ComAutAvaBarra2";
      UN    "PosBarra2Indietro";
      S     "AutBattNotOkInTrasEspul1";
      U     "AutBattNotOkTraslEspul1";
      R     "AutBattNotOkInTrasEspul1";
      NOP   0;
NETWORK
TITLE =Batteria Not Ok Prova Press.1 in Traslata su Espulsore 1

      U     "AutBattNotOkInTrasEspul1";
      U     "ComAutIndBarra2";
      S     "AutBattNotOkTraslEspul1";
      U     "FineCicloEspulPP1";
      R     "AutBattNotOkTraslEspul1";
      NOP   0;
NETWORK
TITLE =Fine Ciclo Espulsore Prova Pressione 1

      U     "Gest Interfac Pneumo 1".dbx170;
      FP    DB100.DBX   11.1;
      S     "FineCicloEspulPP1";
      U     "StartCiloAutBarra2";
      U     "PosBarra2Avanti";
      R     "FineCicloEspulPP1";
      NOP   0;
NETWORK
TITLE =Com Aut Start Ciclo Espulsore Prova Pressione 1

      U     "Gest Interfac Pneumo 1".dbx170;
      U     "AutBattNotOkTraslEspul1";
      U     "ComAutIndBarra2";
      U     "PosBarra2Indietro";
      UN    "FineCicloEspulPP1";
      =     "ComAutStrartEspulPP1";
NETWORK
TITLE =Fine Ciclo Prova Pressione 2

      U(    ;
      U     "Gest Interfac Pneumo 2".dbx165;
      FP    DB100.DBX   11.3;
      ON    "Gest Interfac Pneumo 2".dbx171;
      )     ;
      S     "FineCicloProvaPress2";
      U(    ;
      U     "StartCiloAutBarra2";
      U     "PosBarra2Avanti";
      O     ;
      UN    "Gest Interfac Pneumo 2".dbx161;
      U     E    100.0;
      )     ;
      R     "FineCicloProvaPress2";
      NOP   0;
NETWORK
TITLE =Com Aut Start Ciclo Prova Pressione 2

      U     "Gest Interfac Pneumo 2".dbx162;
      U     "Gest Interfac Pneumo 2".dbx171;
      U     "ComAutIndBarra2";
      UN    "FineCicloProvaPress2";
      =     "ComAutStartProvaPress2";
NETWORK
TITLE =Batteria Not Ok Prova Pressione 2

      U     "FineCicloProvaPress2";
      U     "Gest Interfac Pneumo 2".dbx166;
      S     "AutBattNotOkProvPres2";
      U     "AutBattNotOkInTrasEspul2";
      R     "AutBattNotOkProvPres2";
      NOP   0;
NETWORK
TITLE =Batteria Not Ok Prova Press.2 in Traslazione su Espulsore 2

      U     "AutBattNotOkProvPres2";
      U     "ComAutAvaBarra2";
      UN    "PosBarra2Indietro";
      S     "AutBattNotOkInTrasEspul2";
      U     "AutBattNotOkTraslEspul2";
      R     "AutBattNotOkInTrasEspul2";
      NOP   0;
NETWORK
TITLE =Batteria Not Ok Prova Press.2 in Traslata su Espulsore 2
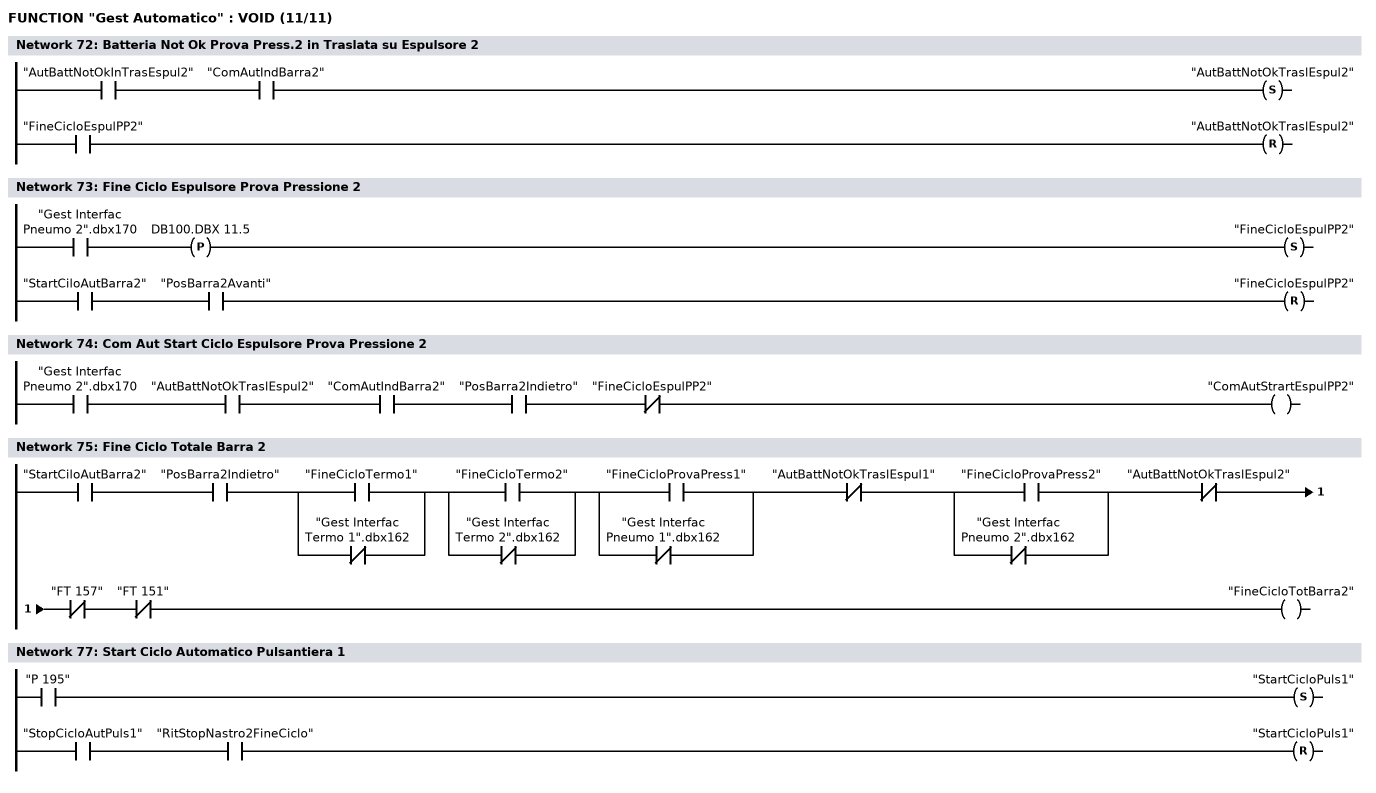
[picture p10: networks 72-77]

      U     "AutBattNotOkInTrasEspul2";
      U     "ComAutIndBarra2";
      S     "AutBattNotOkTraslEspul2";
      U     "FineCicloEspulPP2";
      R     "AutBattNotOkTraslEspul2";
      NOP   0;
NETWORK
TITLE =Fine Ciclo Espulsore Prova Pressione 2

      U     "Gest Interfac Pneumo 2".dbx170;
      FP    DB100.DBX   11.5;
      S     "FineCicloEspulPP2";
      U     "StartCiloAutBarra2";
      U     "PosBarra2Avanti";
      R     "FineCicloEspulPP2";
      NOP   0;
NETWORK
TITLE =Com Aut Start Ciclo Espulsore Prova Pressione 2

      U     "Gest Interfac Pneumo 2".dbx170;
      U     "AutBattNotOkTraslEspul2";
      U     "ComAutIndBarra2";
      U     "PosBarra2Indietro";
      UN    "FineCicloEspulPP2";
      =     "ComAutStrartEspulPP2";
NETWORK
TITLE =Fine Ciclo Totale Barra 2

      U     "StartCiloAutBarra2";
      U     "PosBarra2Indietro";
      U(    ;
      O     "FineCicloTermo1";
      ON    "Gest Interfac Termo 1".dbx162;
      )     ;
      U(    ;
      O     "FineCicloTermo2";
      ON    "Gest Interfac Termo 2".dbx162;
      )     ;
      U(    ;
      O     "FineCicloProvaPress1";
      ON    "Gest Interfac Pneumo 1".dbx162;
      )     ;
      UN    "AutBattNotOkTraslEspul1";
      U(    ;
      O     "FineCicloProvaPress2";
      ON    "Gest Interfac Pneumo 2".dbx162;
      )     ;
      UN    "AutBattNotOkTraslEspul2";
      UN    "FT 157";
      UN    "FT 151";
      =     "FineCicloTotBarra2";
NETWORK
TITLE ======== Automatico Pulsantiera 1 =======

NETWORK
TITLE =Start Ciclo Automatico Pulsantiera 1

      U     "P 195";
      S     "StartCicloPuls1";
      U     "StopCicloAutPuls1";
      U     "RitStopNastro2FineCiclo";
      R     "StartCicloPuls1";
      NOP   0;
NETWORK
TITLE =Stop Ciclo Automatico Pulsantiera 1

      U(    ;
      UN    "P 196";
      S     "StopCicloAutPuls1";
      U     "P 195";
      R     "StopCicloAutPuls1";
      U     "StopCicloAutPuls1";
      )     ;
      UN    "Gest Interfac Pneumo 2".dbx172;
      UN    "FT 151";
      UN    "FT 157";
      L     "Scambio dati OP".TIME_RIT_STOP_NASTRO2;
      SE    "RitStopNastro2FineCiclo";
NETWORK
TITLE =Com Aut Start Nastro 2
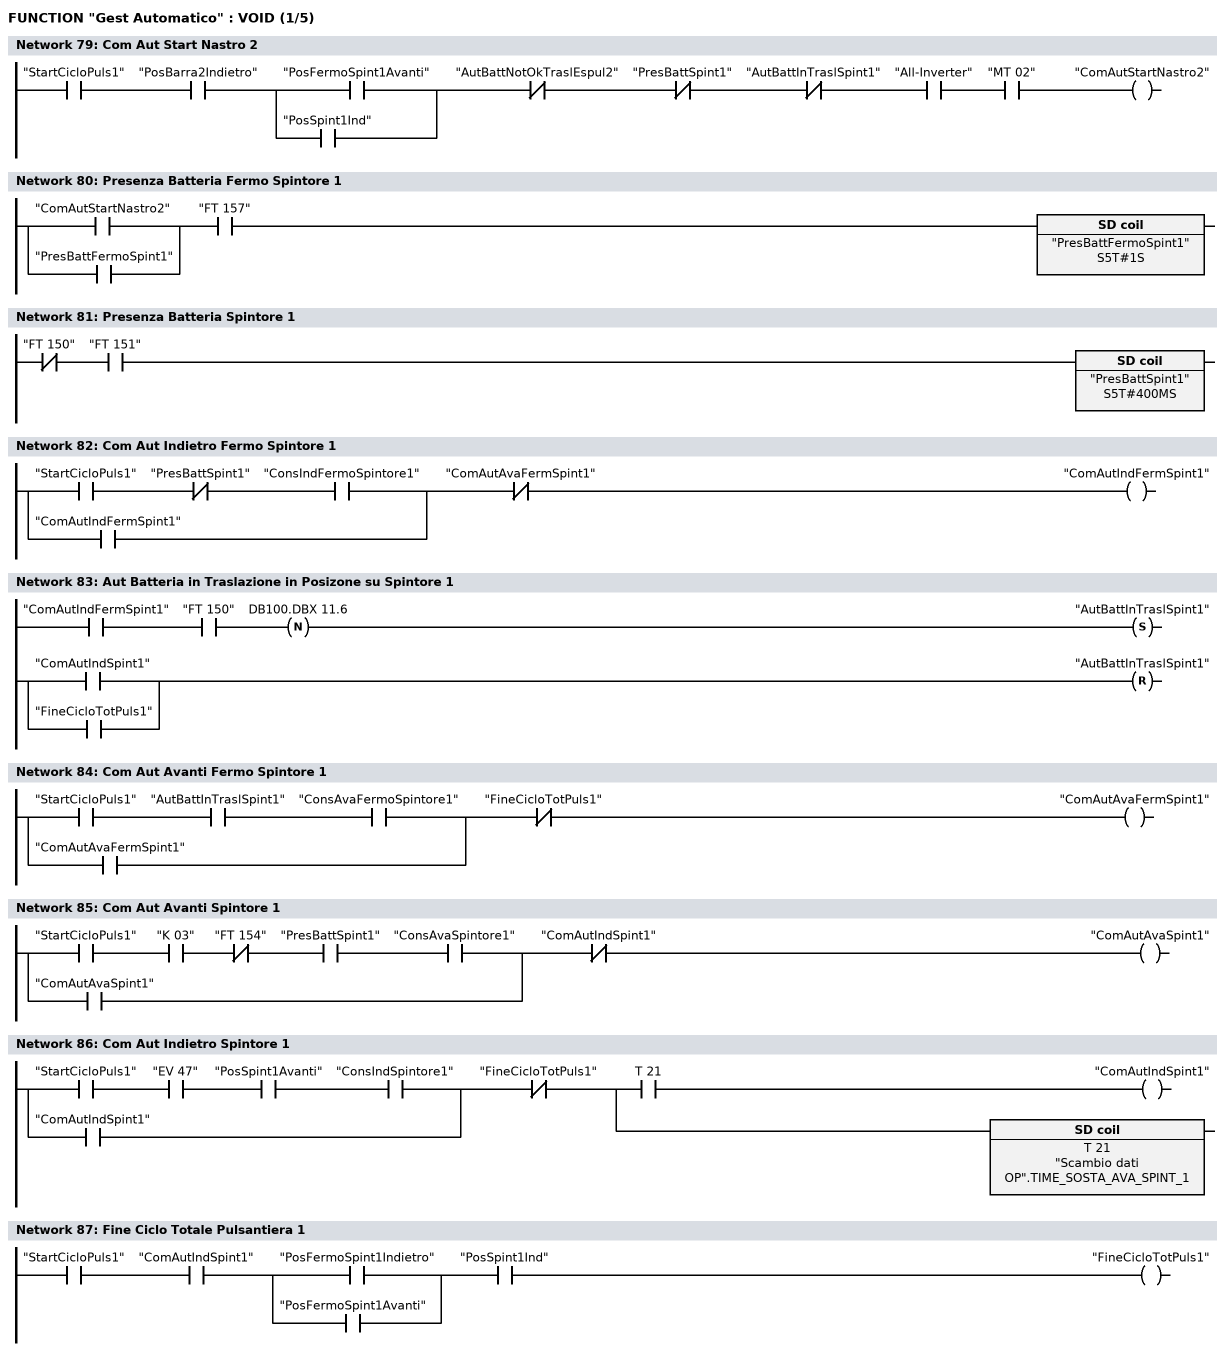
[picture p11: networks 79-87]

      U     "StartCicloPuls1";
      U     "PosBarra2Indietro";
      U(    ;
      O     "PosFermoSpint1Avanti";
      O     "PosSpint1Ind";
      )     ;
      UN    "AutBattNotOkTraslEspul2";
      UN    "PresBattSpint1";
      UN    "AutBattInTraslSpint1";
      U     "All-Inverter";
      U     "MT 02";
      =     "ComAutStartNastro2";
NETWORK
TITLE =Presenza Batteria Fermo Spintore 1

      U(    ;
      O     "ComAutStartNastro2";
      O     "PresBattFermoSpint1";
      )     ;
      U     "FT 157";
      L     S5T#1S;
      SE    "PresBattFermoSpint1";
NETWORK
TITLE =Presenza Batteria Spintore 1

      UN    "FT 150";
      U     "FT 151";
      L     S5T#400MS;
      SE    "PresBattSpint1";
NETWORK
TITLE =Com Aut Indietro Fermo Spintore 1

      U(    ;
      U     "StartCicloPuls1";
      UN    "PresBattSpint1";
      U     "ConsIndFermoSpintore1";
      O     "ComAutIndFermSpint1";
      )     ;
      UN    "ComAutAvaFermSpint1";
      =     "ComAutIndFermSpint1";
NETWORK
TITLE =Aut Batteria in Traslazione in Posizone su Spintore 1

      U     "ComAutIndFermSpint1";
      U     "FT 150";
      FN    DB100.DBX   11.6;
      S     "AutBattInTraslSpint1";
      U(    ;
      O     "ComAutIndSpint1";
      O     "FineCicloTotPuls1";
      )     ;
      R     "AutBattInTraslSpint1";
      NOP   0;
NETWORK
TITLE =Com Aut Avanti Fermo Spintore 1

      U(    ;
      U     "StartCicloPuls1";
      U     "AutBattInTraslSpint1";
      U     "ConsAvaFermoSpintore1";
      O     "ComAutAvaFermSpint1";
      )     ;
      UN    "FineCicloTotPuls1";
      =     "ComAutAvaFermSpint1";
NETWORK
TITLE =Com Aut Avanti Spintore 1

      U(    ;
      U     "StartCicloPuls1";
      U     "K 03";
      UN    "FT 154";
      U     "PresBattSpint1";
      U     "ConsAvaSpintore1";
      O     "ComAutAvaSpint1";
      )     ;
      UN    "ComAutIndSpint1";
      =     "ComAutAvaSpint1";
NETWORK
TITLE =Com Aut Indietro Spintore 1

      U(    ;
      U     "StartCicloPuls1";
      U     "EV 47";
      U     "PosSpint1Avanti";
      U     "ConsIndSpintore1";
      O     "ComAutIndSpint1";
      )     ;
      UN    "FineCicloTotPuls1";
      =     L      0.0;
      U     L      0.0;
      U     T     21;
      =     "ComAutIndSpint1";
      U     L      0.0;
      BLD   102;
      L     "Scambio dati OP".TIME_SOSTA_AVA_SPINT_1;
      SE    T     21;
NETWORK
TITLE =Fine Ciclo Totale Pulsantiera 1

      U     "StartCicloPuls1";
      U     "ComAutIndSpint1";
      U(    ;
      O     "PosFermoSpint1Indietro";
      O     "PosFermoSpint1Avanti";
      )     ;
      U     "PosSpint1Ind";
      =     "FineCicloTotPuls1";
NETWORK
TITLE ======== Automatico Pulsantiera 2 =======

NETWORK
TITLE =Start Ciclo Automatico Pulsantiera 2
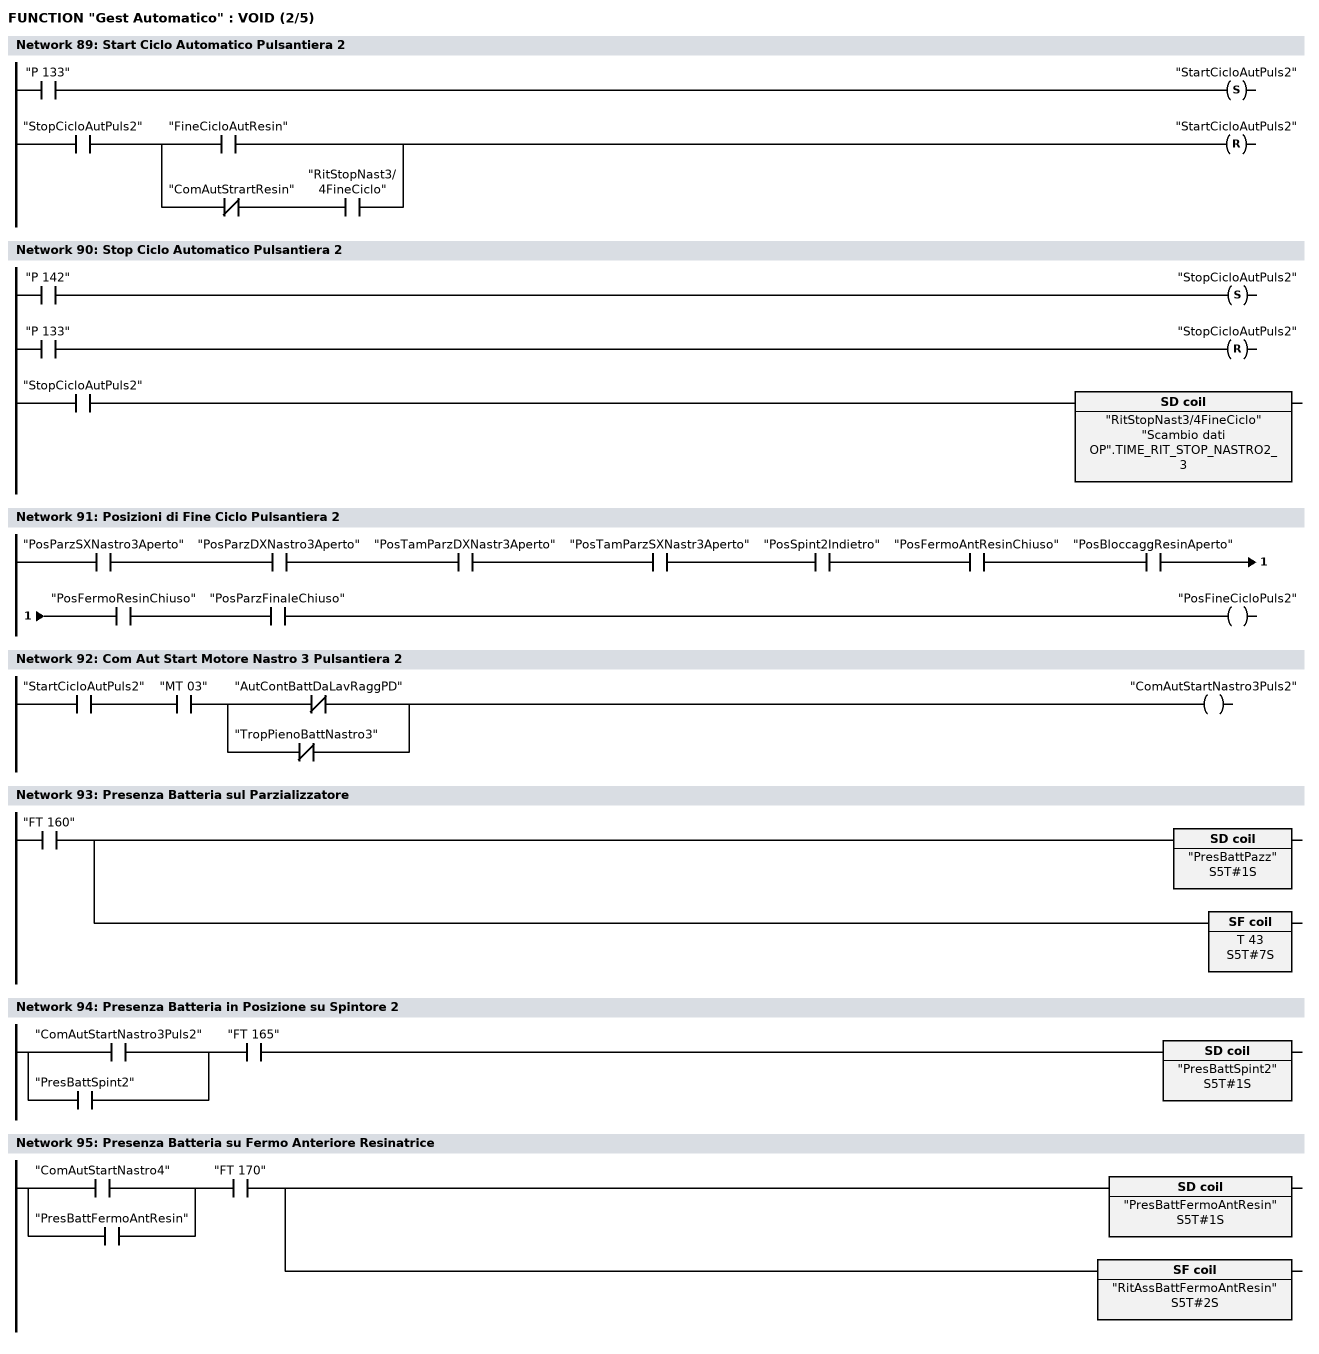
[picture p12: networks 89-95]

      U     "P 133";
      S     "StartCicloAutPuls2";
      U     "StopCicloAutPuls2";
      U(    ;
      O     "FineCicloAutResin";
      O     ;
      UN    "ComAutStrartResin";
      U     "RitStopNast3/4FineCiclo";
      )     ;
      R     "StartCicloAutPuls2";
      NOP   0;
NETWORK
TITLE =Stop Ciclo Automatico Pulsantiera 2

      U     "P 142";
      S     "StopCicloAutPuls2";
      U     "P 133";
      R     "StopCicloAutPuls2";
      U     "StopCicloAutPuls2";
      L     "Scambio dati OP".TIME_RIT_STOP_NASTRO2_3;
      SE    "RitStopNast3/4FineCiclo";
NETWORK
TITLE =Posizioni di Fine Ciclo Pulsantiera 2

      U     "PosParzSXNastro3Aperto";
      U     "PosParzDXNastro3Aperto";
      U     "PosTamParzDXNastr3Aperto";
      U     "PosTamParzSXNastr3Aperto";
      U     "PosSpint2Indietro";
      U     "PosFermoAntResinChiuso";
      U     "PosBloccaggResinAperto";
      U     "PosFermoResinChiuso";
      U     "PosParzFinaleChiuso";
      =     "PosFineCicloPuls2";
NETWORK
TITLE =Com Aut Start Motore Nastro 3 Pulsantiera 2

      U     "StartCicloAutPuls2";
      U     "MT 03";
      U(    ;
      ON    "AutContBattDaLavRaggPD";
      ON    "TropPienoBattNastro3";
      )     ;
      =     "ComAutStartNastro3Puls2";
NETWORK
TITLE =Presenza Batteria sul Parzializzatore

      U     "FT 160";
      L     S5T#1S;
      SE    "PresBattPazz";
      L     S5T#7S;
      SA    T     43;
NETWORK
TITLE =Presenza Batteria in Posizione su Spintore 2

      U(    ;
      O     "ComAutStartNastro3Puls2";
      O     "PresBattSpint2";
      )     ;
      U     "FT 165";
      L     S5T#1S;
      SE    "PresBattSpint2";
NETWORK
TITLE =Presenza Batteria su Fermo Anteriore Resinatrice

      U(    ;
      O     "ComAutStartNastro4";
      O     "PresBattFermoAntResin";
      )     ;
      U     "FT 170";
      L     S5T#1S;
      SE    "PresBattFermoAntResin";
      L     S5T#2S;
      SA    "RitAssBattFermoAntResin";
NETWORK
TITLE =Presenza Batteria in Posizione di Resinatura
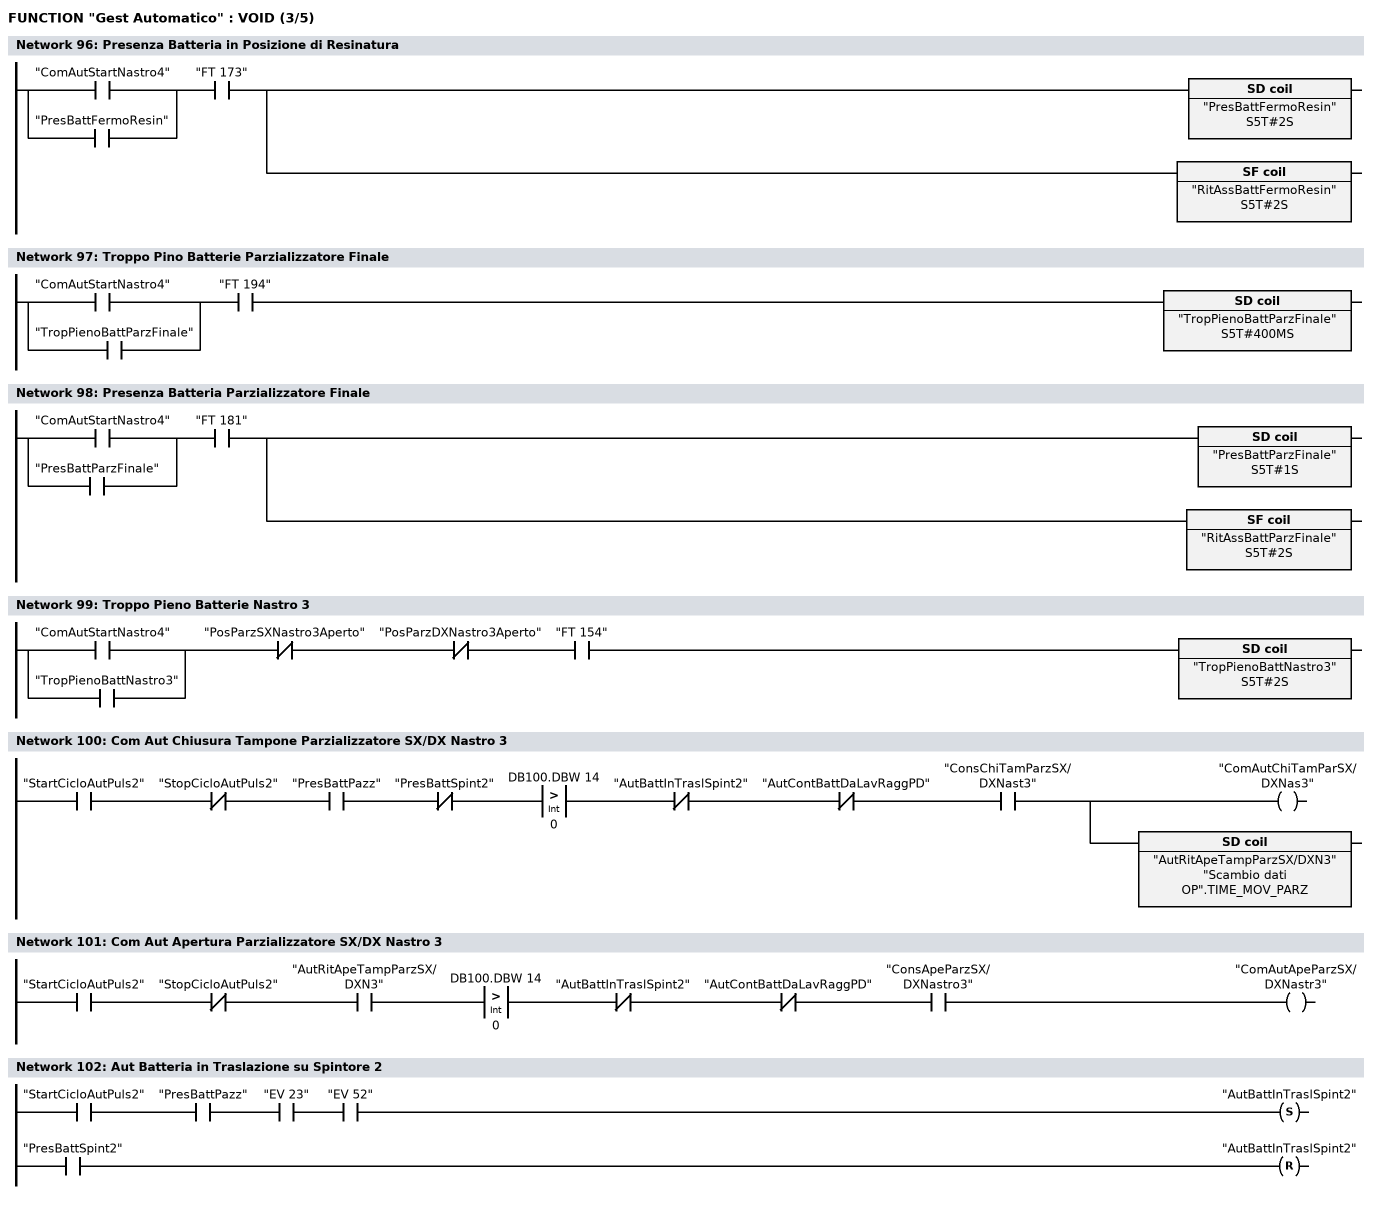
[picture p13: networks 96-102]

      U(    ;
      O     "ComAutStartNastro4";
      O     "PresBattFermoResin";
      )     ;
      U     "FT 173";
      L     S5T#2S;
      SE    "PresBattFermoResin";
      L     S5T#2S;
      SA    "RitAssBattFermoResin";
NETWORK
TITLE =Troppo Pino Batterie Parzializzatore Finale

      U(    ;
      O     "ComAutStartNastro4";
      O     "TropPienoBattParzFinale";
      )     ;
      U     "FT 194";
      L     S5T#400MS;
      SE    "TropPienoBattParzFinale";
NETWORK
TITLE =Presenza Batteria Parzializzatore Finale

      U(    ;
      O     "ComAutStartNastro4";
      O     "PresBattParzFinale";
      )     ;
      U     "FT 181";
      L     S5T#1S;
      SE    "PresBattParzFinale";
      L     S5T#2S;
      SA    "RitAssBattParzFinale";
NETWORK
TITLE =Troppo Pieno Batterie Nastro 3

      U(    ;
      O     "ComAutStartNastro4";
      O     "TropPienoBattNastro3";
      )     ;
      UN    "PosParzSXNastro3Aperto";
      UN    "PosParzDXNastro3Aperto";
      U     "FT 154";
      L     S5T#2S;
      SE    "TropPienoBattNastro3";
NETWORK
TITLE =Com Aut Chiusura Tampone Parzializzatore SX/DX Nastro 3

      U     "StartCicloAutPuls2";
      UN    "StopCicloAutPuls2";
      U     "PresBattPazz";
      UN    "PresBattSpint2";
      U(    ;
      L     DB100.DBW   14;
      L     0;
      >I    ;
      )     ;
      UN    "AutBattInTraslSpint2";
      UN    "AutContBattDaLavRaggPD";
      U     "ConsChiTamParzSX/DXNast3";
      =     "ComAutChiTamParSX/DXNas3";
      L     "Scambio dati OP".TIME_MOV_PARZ;
      SE    "AutRitApeTampParzSX/DXN3";
NETWORK
TITLE =Com Aut Apertura Parzializzatore SX/DX Nastro 3

      U     "StartCicloAutPuls2";
      UN    "StopCicloAutPuls2";
      U     "AutRitApeTampParzSX/DXN3";
      U(    ;
      L     DB100.DBW   14;
      L     0;
      >I    ;
      )     ;
      UN    "AutBattInTraslSpint2";
      UN    "AutContBattDaLavRaggPD";
      U     "ConsApeParzSX/DXNastro3";
      =     "ComAutApeParzSX/DXNastr3";
NETWORK
TITLE =Aut Batteria in Traslazione su Spintore 2

      U     "StartCicloAutPuls2";
      U     "PresBattPazz";
      U     "EV 23";
      U     "EV 52";
      S     "AutBattInTraslSpint2";
      U     "PresBattSpint2";
      R     "AutBattInTraslSpint2";
      NOP   0;
NETWORK
TITLE =Com Aut Chiusura Parzializzatore SX/DX Nastro 3
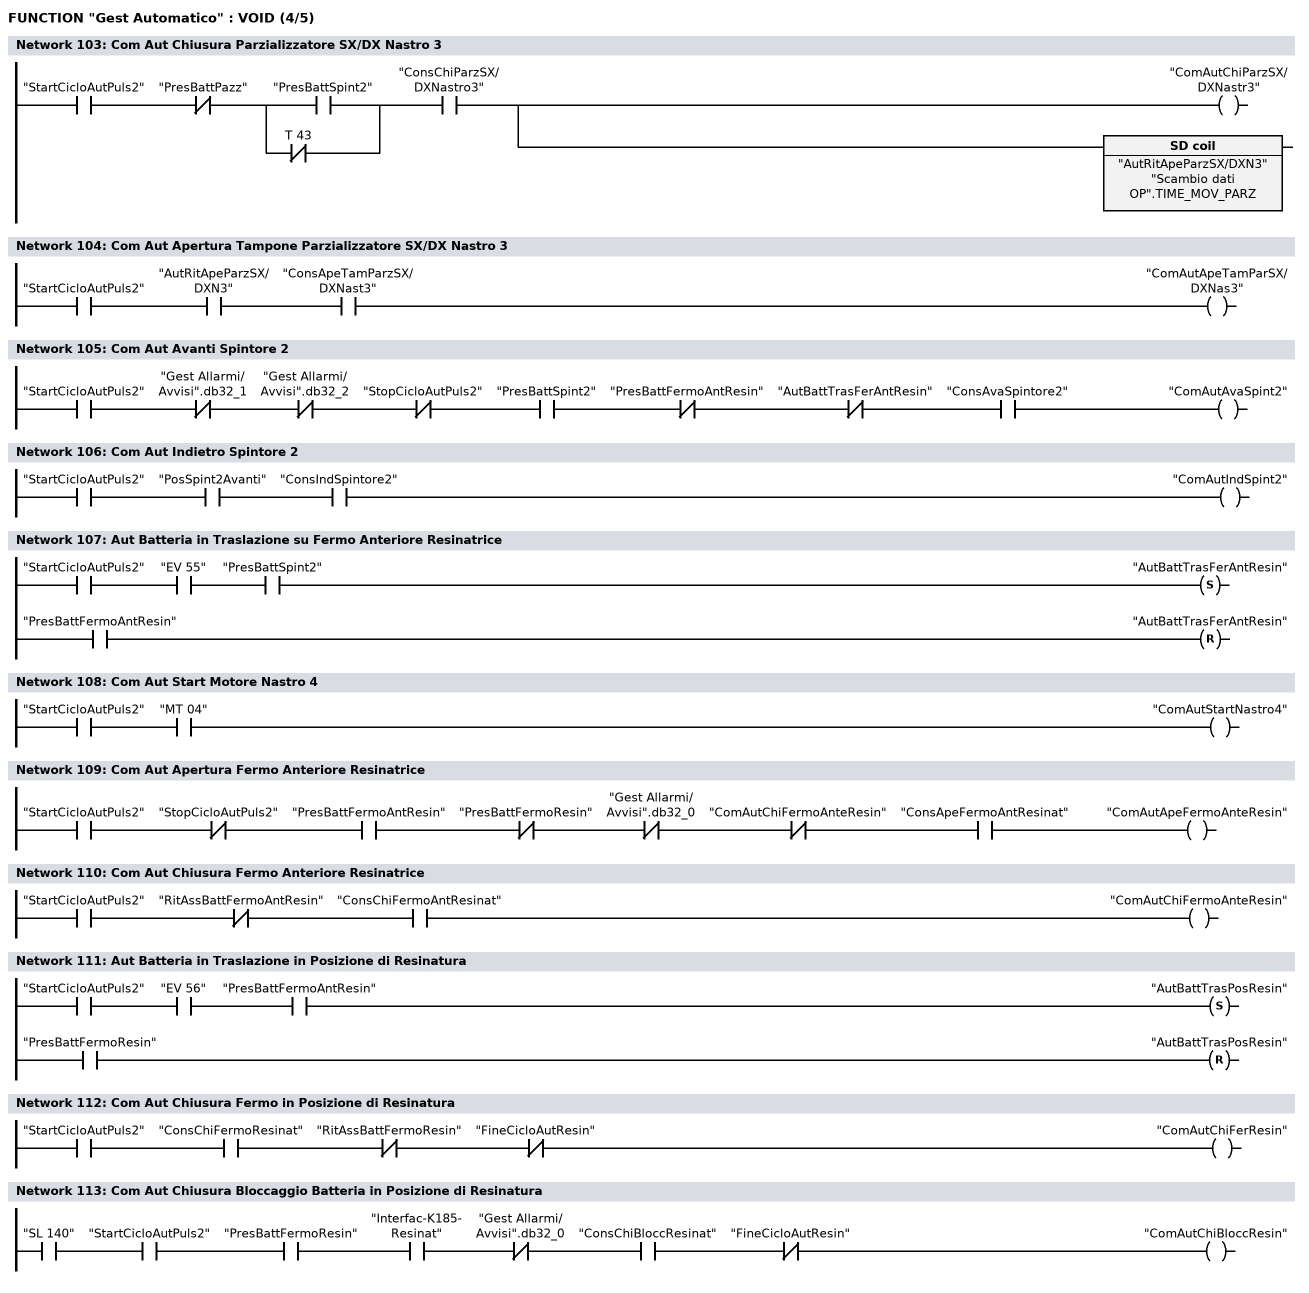
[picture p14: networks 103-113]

      U     "StartCicloAutPuls2";
      UN    "PresBattPazz";
      U(    ;
      O     "PresBattSpint2";
      ON    T     43;
      )     ;
      U     "ConsChiParzSX/DXNastro3";
      =     "ComAutChiParzSX/DXNastr3";
      L     "Scambio dati OP".TIME_MOV_PARZ;
      SE    "AutRitApeParzSX/DXN3";
NETWORK
TITLE =Com Aut Apertura Tampone Parzializzatore SX/DX Nastro 3

      U     "StartCicloAutPuls2";
      U     "AutRitApeParzSX/DXN3";
      U     "ConsApeTamParzSX/DXNast3";
      =     "ComAutApeTamParSX/DXNas3";
NETWORK
TITLE =Com Aut Avanti Spintore 2

      U     "StartCicloAutPuls2";
      UN    "Gest Allarmi/Avvisi".db32_1;
      UN    "Gest Allarmi/Avvisi".db32_2;
      UN    "StopCicloAutPuls2";
      U     "PresBattSpint2";
      UN    "PresBattFermoAntResin";
      UN    "AutBattTrasFerAntResin";
      U     "ConsAvaSpintore2";
      =     "ComAutAvaSpint2";
NETWORK
TITLE =Com Aut Indietro Spintore 2

      U     "StartCicloAutPuls2";
      U     "PosSpint2Avanti";
      U     "ConsIndSpintore2";
      =     "ComAutIndSpint2";
NETWORK
TITLE =Aut Batteria in Traslazione su Fermo Anteriore Resinatrice

      U     "StartCicloAutPuls2";
      U     "EV 55";
      U     "PresBattSpint2";
      S     "AutBattTrasFerAntResin";
      U     "PresBattFermoAntResin";
      R     "AutBattTrasFerAntResin";
      NOP   0;
NETWORK
TITLE =Com Aut Start Motore Nastro 4

      U     "StartCicloAutPuls2";
      U     "MT 04";
      =     "ComAutStartNastro4";
NETWORK
TITLE =Com Aut Apertura Fermo Anteriore Resinatrice

      U     "StartCicloAutPuls2";
      UN    "StopCicloAutPuls2";
      U     "PresBattFermoAntResin";
      UN    "PresBattFermoResin";
      UN    "Gest Allarmi/Avvisi".db32_0;
      UN    "ComAutChiFermoAnteResin";
      U     "ConsApeFermoAntResinat";
      =     "ComAutApeFermoAnteResin";
NETWORK
TITLE =Com Aut Chiusura Fermo Anteriore Resinatrice

      U     "StartCicloAutPuls2";
      UN    "RitAssBattFermoAntResin";
      U     "ConsChiFermoAntResinat";
      =     "ComAutChiFermoAnteResin";
NETWORK
TITLE =Aut Batteria in Traslazione in Posizione di Resinatura

      U     "StartCicloAutPuls2";
      U     "EV 56";
      U     "PresBattFermoAntResin";
      S     "AutBattTrasPosResin";
      U     "PresBattFermoResin";
      R     "AutBattTrasPosResin";
      NOP   0;
NETWORK
TITLE =Com Aut Chiusura Fermo in Posizione di Resinatura

      U     "StartCicloAutPuls2";
      U     "ConsChiFermoResinat";
      UN    "RitAssBattFermoResin";
      UN    "FineCicloAutResin";
      =     "ComAutChiFerResin";
NETWORK
TITLE =Com Aut Chiusura Bloccaggio Batteria in Posizione di Resinatura

      U     "SL 140";
      U     "StartCicloAutPuls2";
      U     "PresBattFermoResin";
      U     "Interfac-K185-Resinat";
      UN    "Gest Allarmi/Avvisi".db32_0;
      U     "ConsChiBloccResinat";
      UN    "FineCicloAutResin";
      =     "ComAutChiBloccResin";
NETWORK
TITLE =Com Aut Start Ciclo Resinatrice
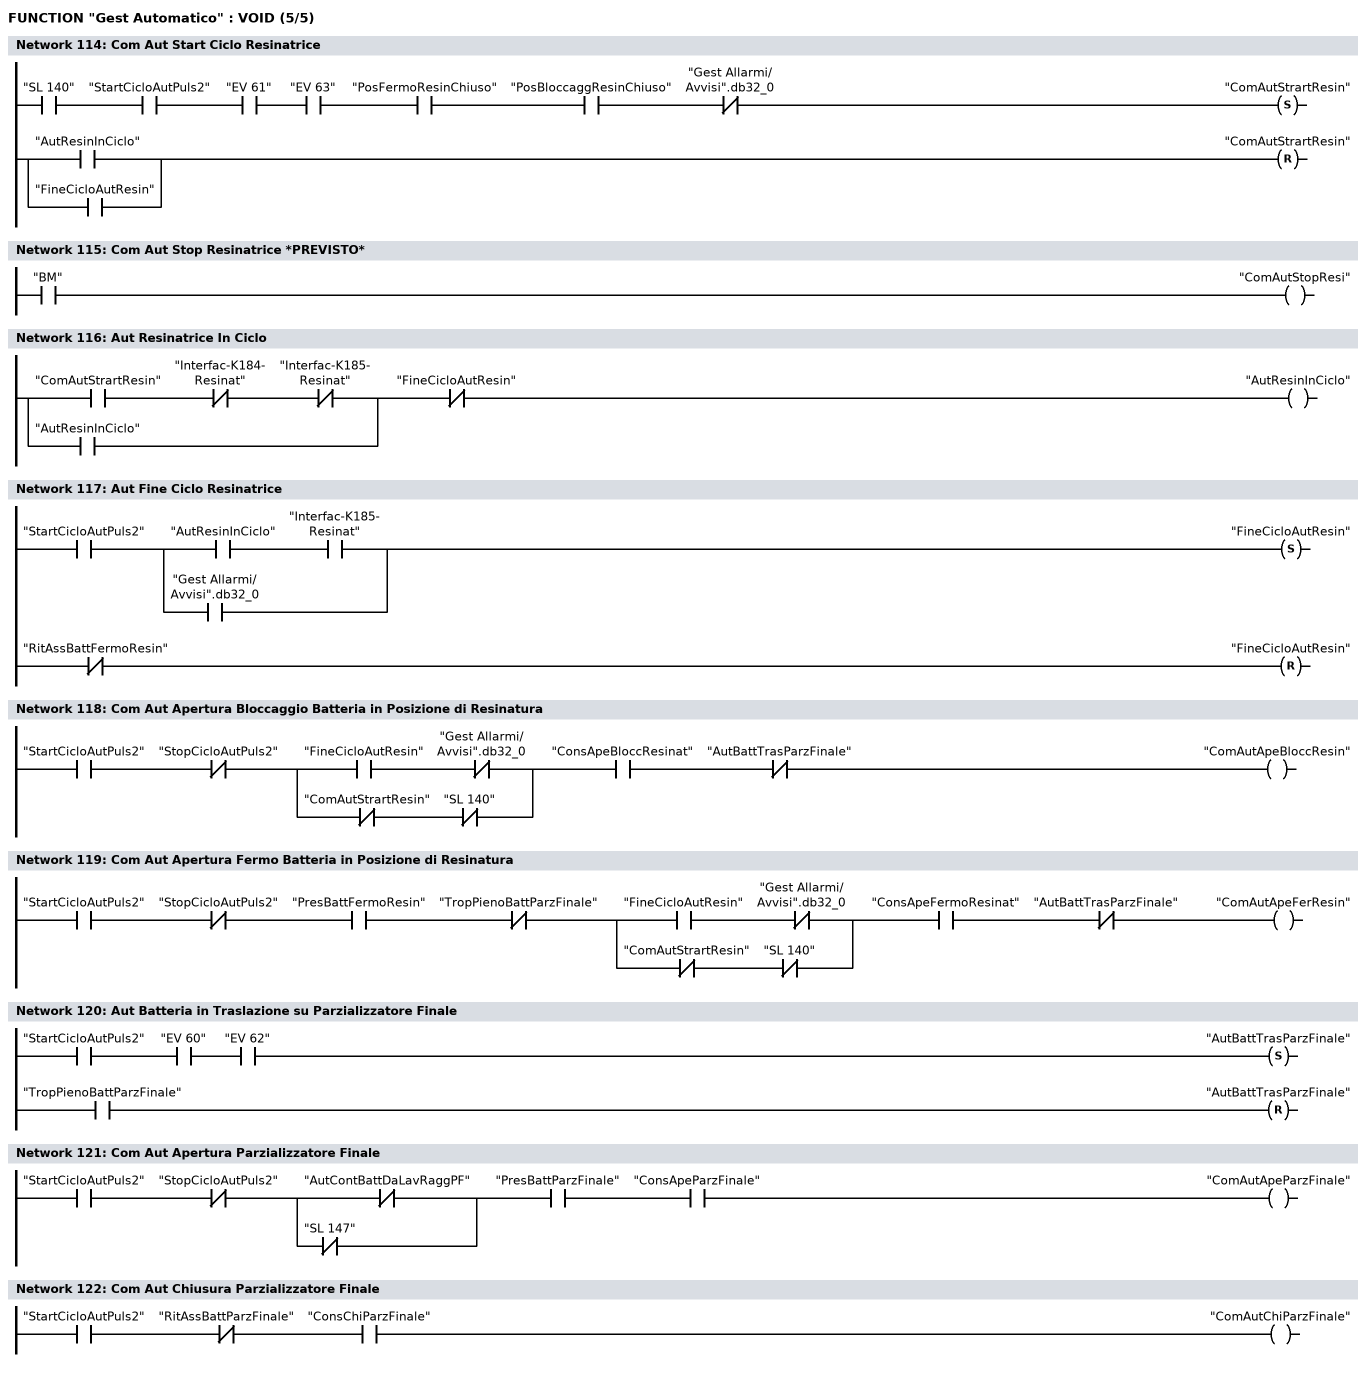
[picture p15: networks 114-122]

      U     "SL 140";
      U     "StartCicloAutPuls2";
      U     "EV 61";
      U     "EV 63";
      U     "PosFermoResinChiuso";
      U     "PosBloccaggResinChiuso";
      UN    "Gest Allarmi/Avvisi".db32_0;
      S     "ComAutStrartResin";
      U(    ;
      O     "AutResinInCiclo";
      O     "FineCicloAutResin";
      )     ;
      R     "ComAutStrartResin";
      NOP   0;
NETWORK
TITLE =Com Aut Stop Resinatrice *PREVISTO*

      U     "BM";
      =     "ComAutStopResi";
NETWORK
TITLE =Aut Resinatrice In Ciclo

      U(    ;
      U     "ComAutStrartResin";
      UN    "Interfac-K184-Resinat";
      UN    "Interfac-K185-Resinat";
      O     "AutResinInCiclo";
      )     ;
      UN    "FineCicloAutResin";
      =     "AutResinInCiclo";
NETWORK
TITLE =Aut Fine Ciclo Resinatrice

      U     "StartCicloAutPuls2";
      U(    ;
      U     "AutResinInCiclo";
      U     "Interfac-K185-Resinat";
      O     "Gest Allarmi/Avvisi".db32_0;
      )     ;
      S     "FineCicloAutResin";
      UN    "RitAssBattFermoResin";
      R     "FineCicloAutResin";
      NOP   0;
NETWORK
TITLE =Com Aut Apertura Bloccaggio Batteria in Posizione di Resinatura

      U     "StartCicloAutPuls2";
      UN    "StopCicloAutPuls2";
      U(    ;
      U     "FineCicloAutResin";
      UN    "Gest Allarmi/Avvisi".db32_0;
      O     ;
      UN    "ComAutStrartResin";
      UN    "SL 140";
      )     ;
      U     "ConsApeBloccResinat";
      UN    "AutBattTrasParzFinale";
      =     "ComAutApeBloccResin";
NETWORK
TITLE =Com Aut Apertura Fermo Batteria in Posizione di Resinatura

      U     "StartCicloAutPuls2";
      UN    "StopCicloAutPuls2";
      U     "PresBattFermoResin";
      UN    "TropPienoBattParzFinale";
      U(    ;
      U     "FineCicloAutResin";
      UN    "Gest Allarmi/Avvisi".db32_0;
      O     ;
      UN    "ComAutStrartResin";
      UN    "SL 140";
      )     ;
      U     "ConsApeFermoResinat";
      UN    "AutBattTrasParzFinale";
      =     "ComAutApeFerResin";
NETWORK
TITLE =Aut Batteria in Traslazione su Parzializzatore Finale

      U     "StartCicloAutPuls2";
      U     "EV 60";
      U     "EV 62";
      S     "AutBattTrasParzFinale";
      U     "TropPienoBattParzFinale";
      R     "AutBattTrasParzFinale";
      NOP   0;
NETWORK
TITLE =Com Aut Apertura Parzializzatore Finale

      U     "StartCicloAutPuls2";
      UN    "StopCicloAutPuls2";
      U(    ;
      ON    "AutContBattDaLavRaggPF";
      ON    "SL 147";
      )     ;
      U     "PresBattParzFinale";
      U     "ConsApeParzFinale";
      =     "ComAutApeParzFinale";
NETWORK
TITLE =Com Aut Chiusura Parzializzatore Finale

      U     "StartCicloAutPuls2";
      UN    "RitAssBattParzFinale";
      U     "ConsChiParzFinale";
      =     "ComAutChiParzFinale";
END_FUNCTION

